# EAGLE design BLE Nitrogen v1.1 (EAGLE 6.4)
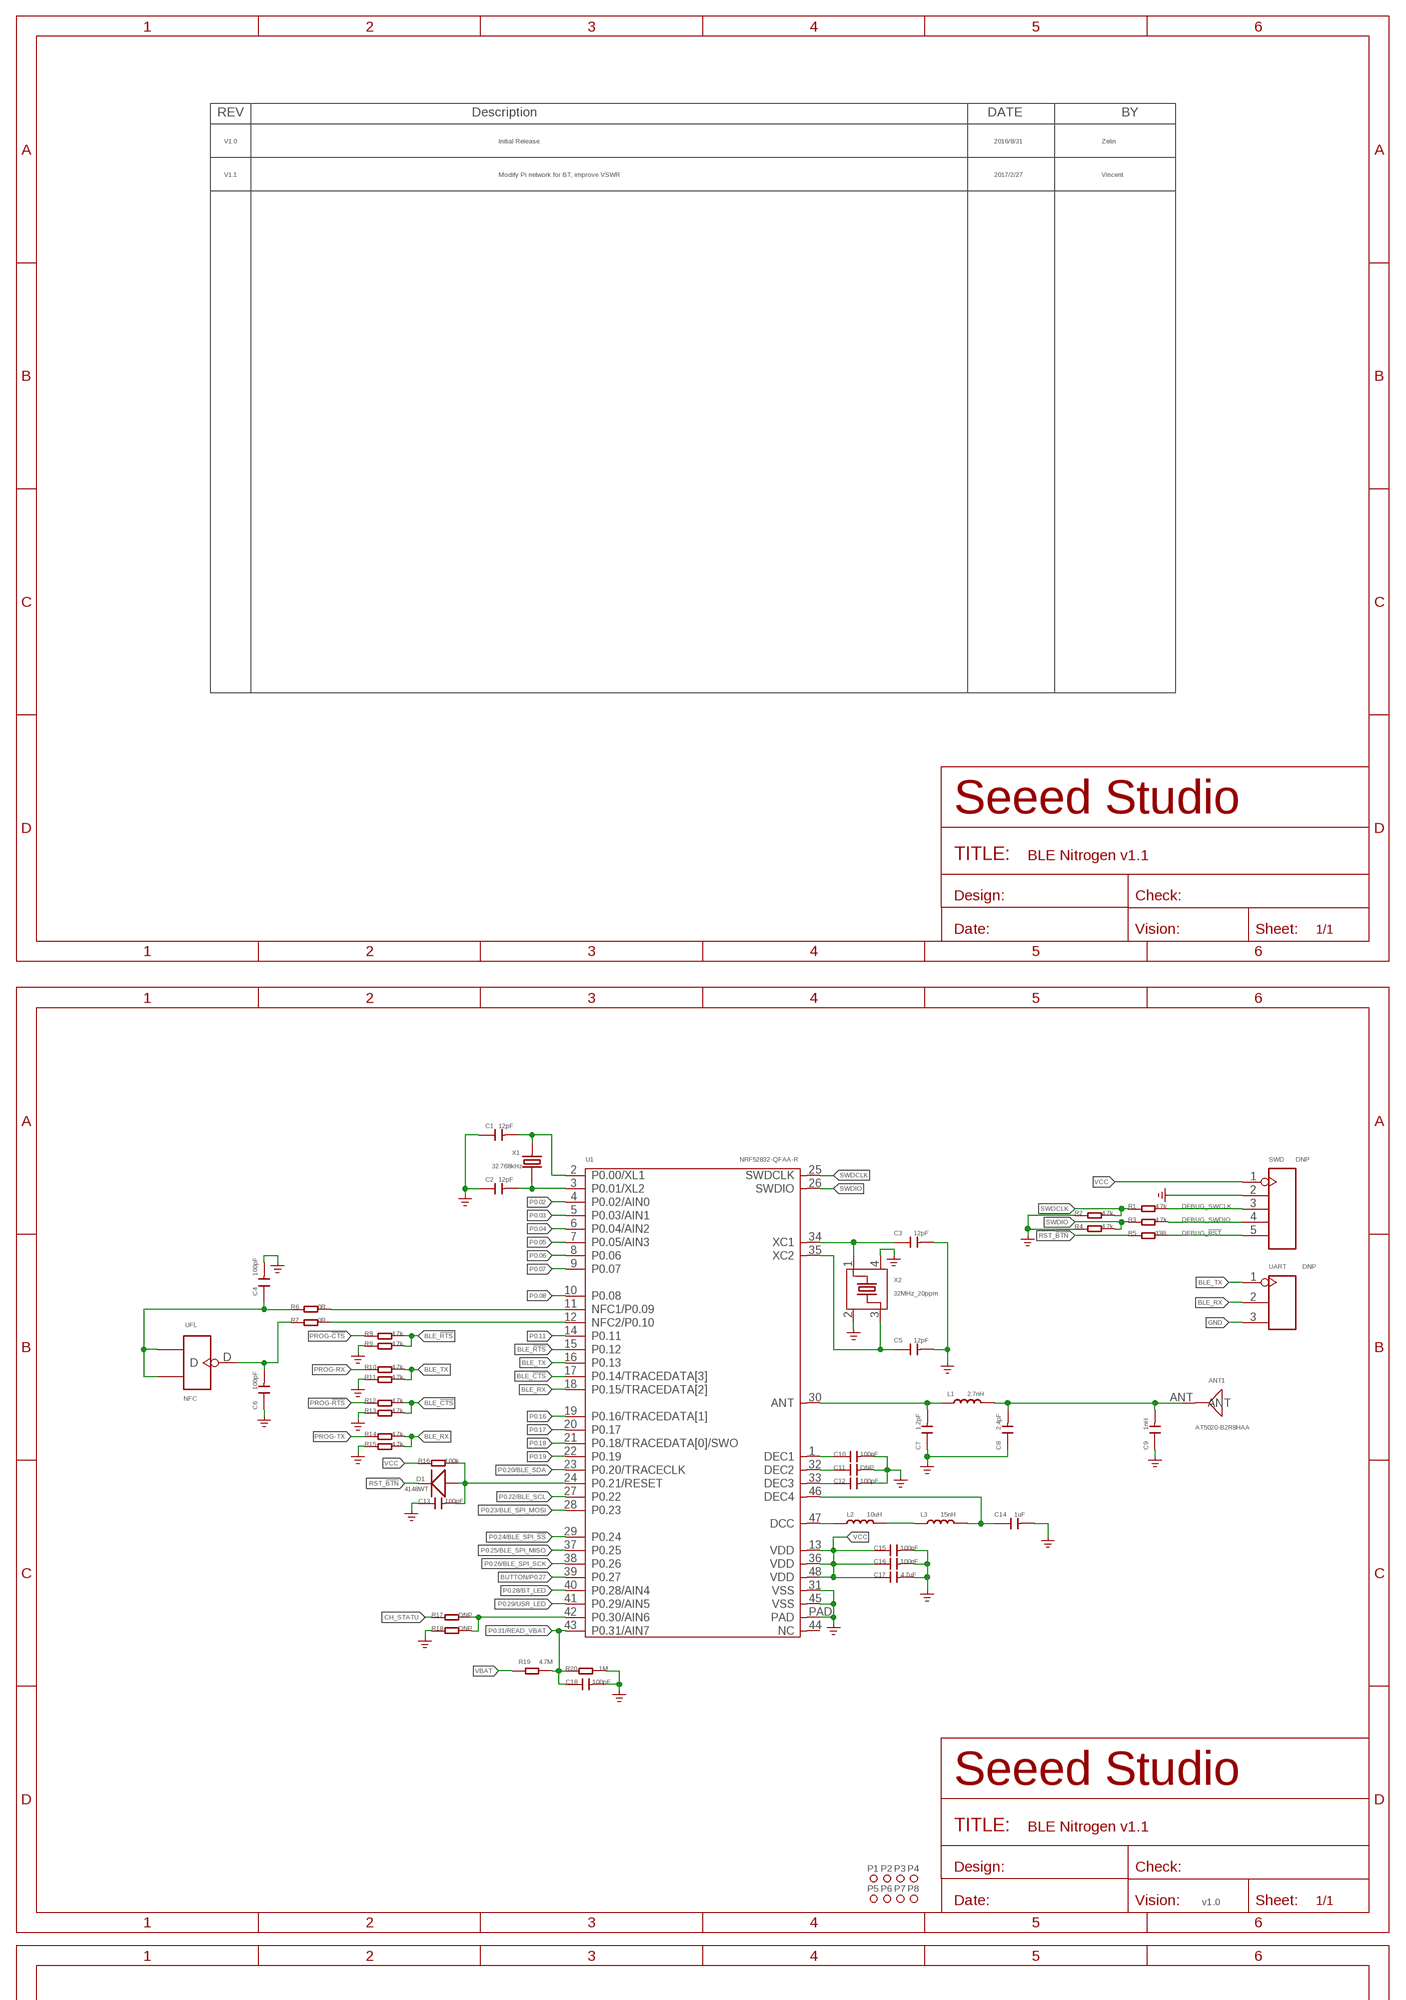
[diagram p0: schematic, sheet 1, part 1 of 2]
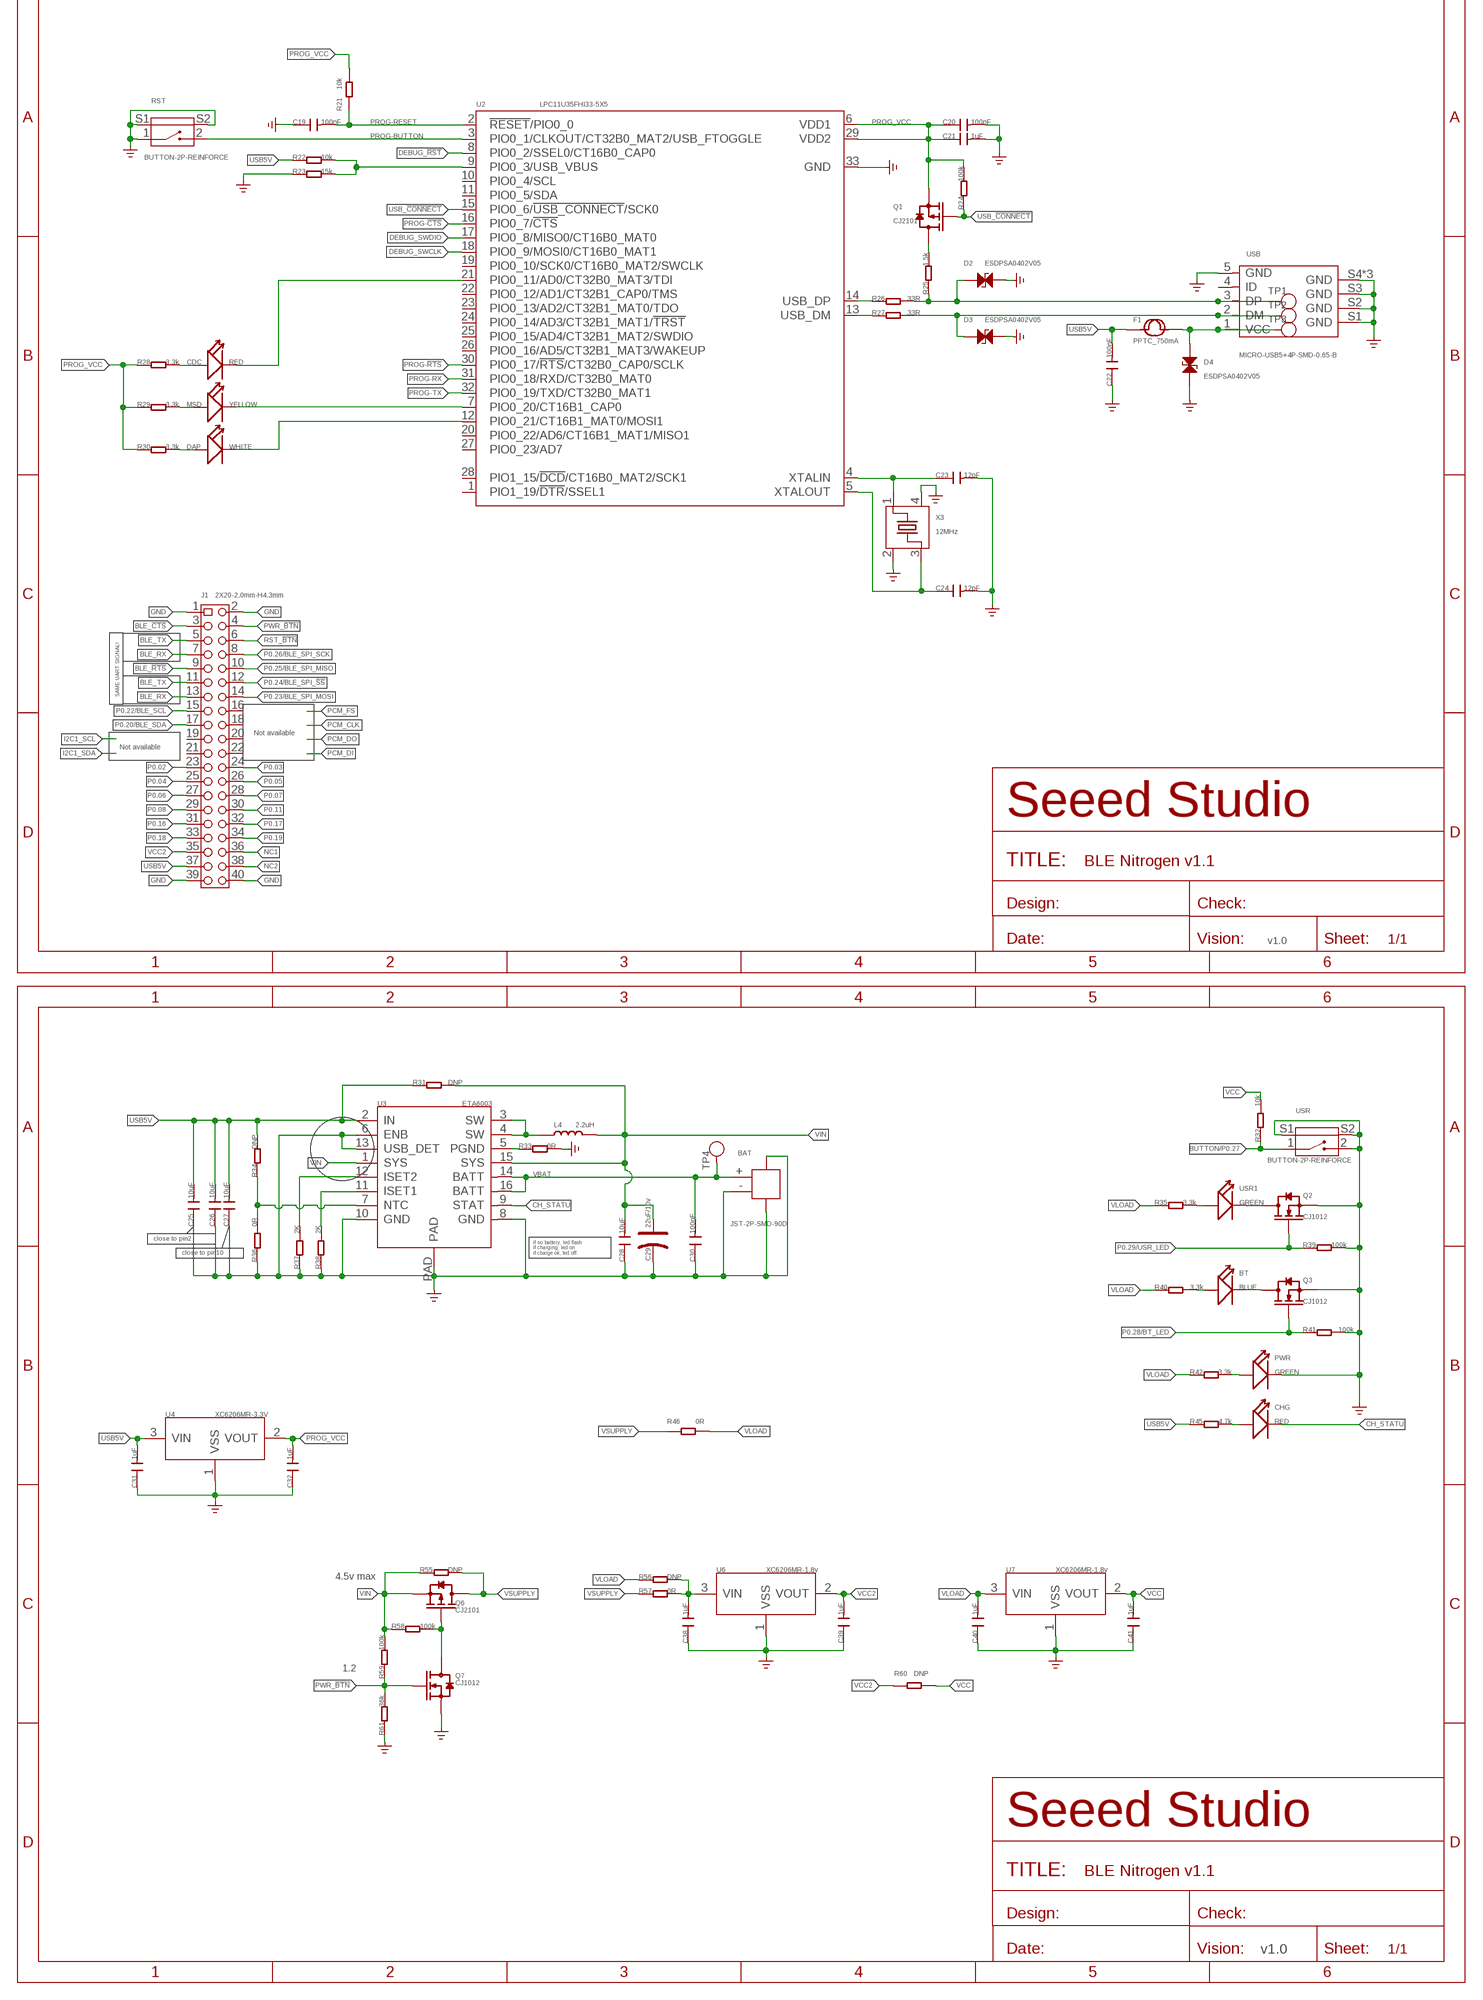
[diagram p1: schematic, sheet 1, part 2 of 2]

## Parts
ANT1  AT5020-B2R8HAA  ANTENNA-AN2051-2.4G  [ANT-SMD2P-5.05X2X1.07MM]
BAT  JST-2P-SMD-90D  JST-2P-SMD'1.0'  [HW2-SMD-1.0-90D]
BT  BLUE  LED'0402'  [LED-0402]
C1  12pF  C-0402  [C0402]
C2  12pF  C-0402  [C0402]
C3  12pF  C-0402  [C0402]
C4  100pF  C-0402  [C0402]
C5  12pF  C-0402  [C0402]
C6  100pF  C-0402  [C0402]
C7  1.2pF  C-0402  [C0402]
C8  2.4pF  C-0402  [C0402]
C9  1nH  C-0402  [C0402]
C10  100nF  C-0402  [C0402]
C11  DNP  C-0402  [C0402]
C12  100pF  C-0402  [C0402]
C13  100pF  C-0402  [C0402]
C14  1uF  C-0402  [C0402]
C15  100nF  C-0402  [C0402]
C16  100nF  C-0402  [C0402]
C17  4.7uF  C-0402  [C0402]
C18  100pF  C-0402  [C0402]
C19  100nF  C-0402  [C0402]
C20  100nF  C-0402  [C0402]
C21  1uF  C-0402  [C0402]
C22  100nF  C-0402  [C0402]
C23  12pF  C-0402  [C0402]
C24  12pF  C-0402  [C0402]
C25  10uF  C-0603  [C0603]
C26  10uF  C-0603  [C0603]
C27  10uF  C-0603  [C0603]
C28  10uF  C-0603  [C0603]
C29  22uF/10v  CAP-POLAR-AVX-A  [AVX-A]
C30  100nF  C-0402  [C0402]
C31  1uF  C-0603  [C0603]
C32  1uF  C-0603  [C0603]
C38  1uF  C-0603  [C0603]
C39  1uF  C-0603  [C0603]
C40  1uF  C-0603  [C0603]
C41  1uF  C-0603  [C0603]
CDC  RED  LED'0402'  [LED-0402]
CHG  RED  LED'0402'  [LED-0402]
D1  4148WT  D'0603'  [SOD523]
D2  ESDPSA0402V05  D-ESD-2P-DOUBLE  [ESD-0402]
D3  ESDPSA0402V05  D-ESD-2P-DOUBLE  [ESD-0402]
D4  ESDPSA0402V05  D-ESD-2P-DOUBLE  [ESD-0402]
DAP  WHITE  LED'0402'  [LED-0402]
F1  PPTC_750mA  FUSE'1206'  [F1206]
J1  2X20-2.0mm-H4.3mm  HEADER-2X20P-2.0  [H2X20-2.0]
L1  2.7nH  L'0402'  [L0402]
L2  10uH  L'0603'  [L0603]
L3  15nH  L'0402'  [L0402]
L4  2.2uH  L'0805'  [L0805]
MSD  YELLOW  LED'0402'  [LED-0402]
NFC  UFL  ANTENNA-U-FL  [U-FL3P-SMD-2.6X2.6X1.0MM]
P1  MARK-1.0'ANNULAR'  [ROUND-MARK-1.0]
P2  MARK-1.0'ANNULAR'  [ROUND-MARK-1.0]
P3  MARK-1.0'ANNULAR'  [ROUND-MARK-1.0]
P4  MARK-1.0'ANNULAR'  [ROUND-MARK-1.0]
P5  MARK-1.0'ANNULAR'  [ROUND-MARK-1.0]
P6  MARK-1.0'ANNULAR'  [ROUND-MARK-1.0]
P7  MARK-1.0'ANNULAR'  [ROUND-MARK-1.0]
P8  MARK-1.0'ANNULAR'  [ROUND-MARK-1.0]
PWR  GREEN  LED'0402'  [LED-0402]
Q1  CJ2101  MOSFET-P-SOT323  [SOT323]
Q2  CJ1012  MOSFET-N-SOT523  [SOT523]
Q3  CJ1012  MOSFET-N-SOT523  [SOT523]
Q6  CJ2101  MOSFET-P-SOT323  [SOT323]
Q7  CJ1012  MOSFET-N-SOT523  [SOT523]
R1  4.7k  R-0402  [R0402]
R2  4.7k  R-0402  [R0402]
R3  4.7k  R-0402  [R0402]
R4  4.7k  R-0402  [R0402]
R5  33R  R-0402  [R0402]
R6  0R  R-0402  [R0402]
R7  0R  R-0402  [R0402]
R8  4.7k  R-0402  [R0402]
R9  4.7k  R-0402  [R0402]
R10  4.7k  R-0402  [R0402]
R11  4.7k  R-0402  [R0402]
R12  4.7k  R-0402  [R0402]
R13  4.7k  R-0402  [R0402]
R14  4.7k  R-0402  [R0402]
R15  4.7k  R-0402  [R0402]
R16  100k  R-0402  [R0402]
R17  DNP  R-0402  [R0402]
R18  DNP  R-0402  [R0402]
R19  4.7M  R-0402  [R0402]
R20  1M  R-0402  [R0402]
R21  10k  R-0402  [R0402]
R22  10k  R-0402  [R0402]
R23  15k  R-0402  [R0402]
R24  100k  R-0402  [R0402]
R25  1.5k  R-0402  [R0402]
R26  33R  R-0402  [R0402]
R27  33R  R-0402  [R0402]
R28  3.3k  R-0402  [R0402]
R29  3.3k  R-0402  [R0402]
R30  3.3k  R-0402  [R0402]
R31  DNP  R-0402  [R0402]
R32  10k  R-0402  [R0402]
R33  0R  R-0402  [R0402]
R34  DNP  R-0402  [R0402]
R35  3.3k  R-0402  [R0402]
R36  0R  R-0402  [R0402]
R37  2K  R-0402  [R0402]
R38  2K  R-0402  [R0402]
R39  100k  R-0402  [R0402]
R40  3.3k  R-0402  [R0402]
R41  100k  R-0402  [R0402]
R42  3.3k  R-0402  [R0402]
R45  4.7k  R-0402  [R0402]
R46  0R  R-0603  [R0603]
R55  DNP  R-0402  [R0402]
R56  DNP  R-0402  [R0402]
R57  0R  R-0402  [R0402]
R58  100k  R-0402  [R0402]
R59  100k  R-0402  [R0402]
R60  DNP  R-0402  [R0402]
R61  36k  R-0402  [R0402]
RST  BUTTON-2P-REINFORCE  [4P-SMD-4.7X3.5X1.8]
SWD  DNP  HEADER-5P-2.54  [H5-2.54]
TP1  DP  TEST-POINT'4545'  [TP-D45MIL]
TP2  DM  TEST-POINT'4545'  [TP-D45MIL]
TP3  VBUS  TEST-POINT'4545'  [TP-D45MIL]
TP4  VBAT  TEST-POINT'4545'  [TP-D45MIL]
U1  NRF52832-QFAA-R  NRF52832  [QFN48-6X6MM]
U2  LPC11U35FHI33-5X5  [HVQFN33]
U3  ETA6003  PMIC-ETA6003  [QFN16G-0.5-3X3MM]
U4  XC6206MR-3.3V  XC6206MR  [SOT23]
U6  XC6206MR-1.8v  XC6206MR  [SOT23]
U7  XC6206MR-1.8v  XC6206MR  [SOT23]
UART  DNP  HEADER-3P-2.54  [H3-2.54]
USB  MICRO-USB5+4P-SMD-0.65-B  MICRO-USB5+4P'5+4P'  [MICRO-USB5+4P-SMD-0.65-B]
USR  BUTTON-2P-REINFORCE  [4P-SMD-4.7X3.5X1.8]
USR1  GREEN  LED'0402'  [LED-0402]
X1  32.768kHz  CRYSTAL-3215  [2P-SMD-3.2X1.5]
X2  32MHz_20ppm  CRYSTAL-4P  [X4-SMD-3.2X2.5X0.7MM]
X3  12MHz  CRYSTAL-4P  [X4-SMD-3.2X2.5X0.7MM]

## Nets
!RESET: C13.2 D1.+ R16.2 U1.24(P0.21/RESET)
BLE_!CTS: J1.3 R12.2 R13.2 U1.17(P0.14/TRACEDATA[3])
BLE_!RTS: J1.9 R8.2 R9.2 U1.15(P0.12)
BLE_RX: J1.7 J1.13 R14.2 R15.2 U1.18(P0.15/TRACEDATA[2]) UART.2
BLE_TX: J1.5 J1.11 R10.2 R11.2 U1.16(P0.13) UART.1
BUTTON/P0.27: R32.1 U1.39(P0.27) USR.1
CH_STATU: CHG.- R17.1 U3.9(STAT)
DEBUG_!RST: R5.2 SWD.5 U2.8(PIO0_2/SSEL0/CT16B0_CAP0)
DEBUG_SWCLK: R1.2 SWD.3 U2.18(PIO0_9/MOSI0/CT16B0_MAT1)
DEBUG_SWDIO: R3.2 SWD.4 U2.17(PIO0_8/MISO0/CT16B0_MAT0)
GND: BAT.3 BAT.4 BAT.- C1.1 C2.1 C3.2 C4.2 C5.2 C6.1 C7.1 C8.1 C9.1 C10.2 C11.2 C12.2 C13.1 C14.2 C15.2 C16.2 C17.2 C18.2 C19.1 C20.2 C21.2 C22.1 C23.2 C24.2 C25.1 C26.1 C27.1 C28.1 C29.- C30.1 C31.1 C32.1 C38.1 C39.1 C40.1 C41.1 D2.2 D3.2 D4.1 J1.1 J1.2 J1.39 J1.40 PWR.- Q2.2(S) Q3.2(S) Q7.2(S) R2.1 R4.1 R9.1 R11.1 R13.1 R15.1 R18.1 R20.2 R23.1 R33.2 R36.1 R37.1 R38.1 R39.2 R41.2 R61.1 RST.1 RST.S1 RST.S2 SWD.2 U1.31(VSS) U1.45(VSS) U1.PAD U2.33(GND) U3.6(ENB) U3.8(GND) U3.10(GND) U3.13(USB_DET) U3.PAD U4.1(VSS) U6.1(VSS) U7.1(VSS) UART.3 USB.5(GND) USB.S1(GND) USB.S2(GND) USB.S3(GND) USB.S4(GND) USB.S5(GND) USB.S6(GND) USR.2 USR.S1 USR.S2 X2.2 X2.4 X3.2 X3.4 ; supply symbol labelled GND_POWER
N$1: C4.1 NFC.GND1 NFC.GND2 R6.1
N$2: C23.1 U2.4(XTALIN) X3.1
N$3: C14.1 L3.2 U1.46(DEC4)
N$4: C24.1 U2.5(XTALOUT) X3.3
N$5: L2.1 U1.47(DCC)
N$6: R26.1 U2.14(USB_DP)
N$7: R27.1 U2.13(USB_DM)
N$8: D2.1 R25.1 R26.2 TP1.T USB.3(DP)
N$9: CHG.+ R45.2
N$10: Q6.1(G) Q7.3(D) R58.2
N$11: D3.1 R27.2 TP2.T USB.2(DM)
N$12: C1.2 U1.2(P0.00/XL1) X1.2
N$13: C2.2 U1.3(P0.01/XL2) X1.1
N$14: C3.1 U1.34(XC1) X2.1
N$15: C5.1 U1.35(XC2) X2.3
N$16: CDC.- U2.21(PIO0_11/AD0/CT32B0_MAT3/TDI)
N$17: C6.2 NFC.D R7.1
N$18: R6.2 U1.11(NFC1/P0.09)
N$19: C10.1 U1.1(DEC1)
N$20: C11.1 U1.32(DEC2)
N$21: C12.1 U1.33(DEC3)
N$22: R7.2 U1.12(NFC2/P0.10)
N$25: C7.2 L1.1 U1.30(ANT)
N$26: ANT1.ANT C8.2 C9.2 L1.2
N$28: C38.2 R56.2 R57.2 U6.3(VIN)
N$32: L2.2 L3.1
N$33: R35.2 USR1.+
N$34: BT.+ R40.2
N$35: Q2.3(D) USR1.-
N$36: BT.- Q3.3(D)
N$39: Q1.3(D) R25.2
N$40: D4.2 F1.2 TP3.T USB.1(VCC)
N$41: R22.2 R23.2 U2.9(PIO0_3/USB_VBUS)
N$42: CDC.+ R28.2
N$43: DAP.+ R30.2
N$44: MSD.+ R29.2
N$46: MSD.- U2.7(PIO0_20/CT16B1_CAP0)
N$47: DAP.- U2.12(PIO0_21/CT16B1_MAT0/MOSI1)
N$58: PWR.+ R42.2
N$84: L4.1 U3.3(SW) U3.4(SW)
N$88: R34.1 R36.2 U3.7(NTC)
N$89: R38.2 U3.11(ISET1)
N$90: R37.2 U3.12(ISET2)
N$91: R33.1 U3.5(PGND)
NC1: J1.36
NC2: J1.38
P0.02: J1.23 U1.4(P0.02/AIN0)
P0.03: J1.24 U1.5(P0.03/AIN1)
P0.04: J1.25 U1.6(P0.04/AIN2)
P0.05: J1.26 U1.7(P0.05/AIN3)
P0.06: J1.27 U1.8(P0.06)
P0.07: J1.28 U1.9(P0.07)
P0.08: J1.29 U1.10(P0.08)
P0.11: J1.30 U1.14(P0.11)
P0.16: J1.31 U1.19(P0.16/TRACEDATA[1])
P0.17: J1.32 U1.20(P0.17)
P0.18: J1.33 U1.21(P0.18/TRACEDATA[0]/SWO)
P0.19: J1.34 U1.22(P0.19)
P0.20/BLE_SDA: J1.17 U1.23(P0.20/TRACECLK)
P0.22/BLE_SCL: J1.15 U1.27(P0.22)
P0.23/BLE_SPI_MOSI: J1.14 U1.28(P0.23)
P0.24/BLE_SPI_!SS: J1.12 U1.29(P0.24)
P0.25/BLE_SPI_MISO: J1.10 U1.37(P0.25)
P0.26/BLE_SPI_SCK: J1.8 U1.38(P0.26)
P0.28/BT_LED: Q3.1(G) R41.1 U1.40(P0.28/AIN4)
P0.29/USR_LED: Q2.1(G) R39.1 U1.41(P0.29/AIN5)
P0.30/AIN6: R17.2 R18.2 U1.42(P0.30/AIN6)
P0.31/READ_VBAT: C18.1 R19.2 R20.1 U1.43(P0.31/AIN7)
PROG-!CTS!: R8.1 U2.16(PIO0_7/!CTS!)
PROG-!RTS!: R12.1 U2.30(PIO0_17/!RTS!/CT32B0_CAP0/SCLK)
PROG-BUTTON: RST.2 U2.3(PIO0_1/CLKOUT/CT32B0_MAT2/USB_FTOGGLE)
PROG-RESET: C19.2 R21.1 U2.2(!RESET!/PIO0_0)
PROG-RX: R10.1 U2.31(PIO0_18/RXD/CT32B0_MAT0)
PROG-TX: R14.1 U2.32(PIO0_19/TXD/CT32B0_MAT1)
PROG_VCC: C20.1 C21.1 C32.2 Q1.2(S) R21.2 R24.2 R28.1 R29.1 R30.1 U2.6(VDD1) U2.29(VDD2) U4.2(VOUT)
PWR_!BTN: J1.4 Q7.1(G) R59.1 R61.2
RST_!BTN: D1.- J1.6 R5.1
SWDCLK: R1.1 R2.2 U1.25(SWDCLK)
SWDIO: R3.1 R4.2 U1.26(SWDIO)
USB5V: C22.2 C25.2 C26.2 C27.2 C31.2 F1.1 J1.37 R22.1 R31.1 R34.2 R45.1 U3.2(IN) U4.3(VIN)
USB_!CONNECT!: Q1.1(G) R24.1 U2.15(PIO0_6/!USB_CONNECT!/SCK0)
VBAT: BAT.+ C30.2 R19.1 TP4.T U3.14(BATT) U3.16(BATT)
VCC: C15.1 C16.1 C17.1 C41.2 R16.1 R32.2 R60.1 SWD.1 U1.13(VDD) U1.36(VDD) U1.48(VDD) U7.2(VOUT)
VCC2: C39.2 J1.35 R60.2 U6.2(VOUT)
VIN: C28.2 C29.+ L4.2 Q6.2(S) R31.2 R55.1 R58.1 R59.2 U3.1(SYS) U3.15(SYS)
VLOAD: C40.2 R35.1 R40.1 R42.1 R46.2 R56.1 U7.3(VIN)
VSUPPLY: Q6.3(D) R46.1 R55.2 R57.1
Unconnected: J1.16 J1.18 J1.19 J1.20 J1.21 J1.22 U1.44(NC) U2.1(PIO1_19/!DTR!/SSEL1) U2.10(PIO0_4/SCL) U2.11(PIO0_5/SDA) U2.19(PIO0_10/SCK0/CT16B0_MAT2/SWCLK) U2.20(PIO0_22/AD6/CT16B1_MAT1/MISO1) U2.22(PIO0_12/AD1/CT32B1_CAP0/TMS) U2.23(PIO0_13/AD2/CT32B1_MAT0/TDO) U2.24(PIO0_14/AD3/CT32B1_MAT1/!TRST!) U2.25(PIO0_15/AD4/CT32B1_MAT2/SWDIO) U2.26(PIO0_16/AD5/CT32B1_MAT3/WAKEUP) U2.27(PIO0_23/AD7) U2.28(PIO1_15/!DCD!/CT16B0_MAT2/SCK1) USB.4(ID)

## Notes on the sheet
- V1.0 | Initial Release. | 2016/8/31 | Zelin
- V1.1 | Modify Pi network for BT, improve VSWR | 2017/2/27 | Vincent
- v1.0
- SAME UART SIGNAL!
- Not available
- Not available
- v1.0
- close to pin2
- close to pin10
- if no battery, led flash.
  if charging, led on.
  if charge ok, led off.
- 4.5v max
- 1.2
- v1.0

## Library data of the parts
ANT1 = Connector-new:ANTENNA-AN2051-2.4G: Multilayer Chip Antenna for 2.4GHz Wireless Communication
BAT = Connector-update:JST-2P-SMD: 2P-SMD-1.0-90D:320110054;2P-SMD-2.0-90D:320110026
BT CDC CHG DAP MSD PWR USR1 = Discrete:LED*
C1-C28 C30-C32 C38-C41 = Discrete:C*: Ceramic Capacitors
C29 = Discrete-new:CAP-POLAR: Electrolytic Capacitors,Tantalum Capacitors and Super Capacitors
D1 = Discrete:D*
D2-D4 = Discrete-new:D-ESD-2P-DOUBLE
F1 = Discrete:FUSE
J1 = Connector-update:HEADER-2X20P-2.0
L1-L4 = Discrete:L*
NFC = Connector-update:ANTENNA-U-FL: 320110048
P1-P8 = Discrete-new:MARK-1.0; PARTNO: DNP
Q1 Q6 = Discrete:MOSFET-P
Q2 Q3 Q7 = Discrete:MOSFET-N: IRLL014: http://www.vishay.com/docs/91319/sihll014.pdf
R1-R42 R45 R46 R55-R61 = Discrete:R*
RST USR = Discrete:BUTTON-2P-REINFORCE: TS-1188E http://www.best-dz.com/?thread-374-2.html SMD Button
SWD = Connector-update:HEADER-5P
TP1-TP4 = Discrete-new:TEST-POINT; PARTNO: DNP
U1 = AMLib:NRF52832
U2 = AMLib:LPC11U35FHI33
U3 = AMLib_New:PMIC-ETA6003: 2.5A,3MHZ Switching Charger with Dynamic Power Path Management
U4 U6 U7 = IC:XC6206: LOW ESR Cap.Compatible Positive Voltage Regulators
UART = Connector-update:HEADER-3P
USB = Connector-new:MICRO-USB5+4P: 5+4P-SMD-0.65-B:320010000;5+2P-SMD-0.65-AB:340032001
X1 = Discrete:CRYSTAL*: CRYSTAL
X2 X3 = Discrete-new:CRYSTAL-4P

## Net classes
0 default: width 0.127 mm, drill 0.203 mm, clearance 0.152 mm

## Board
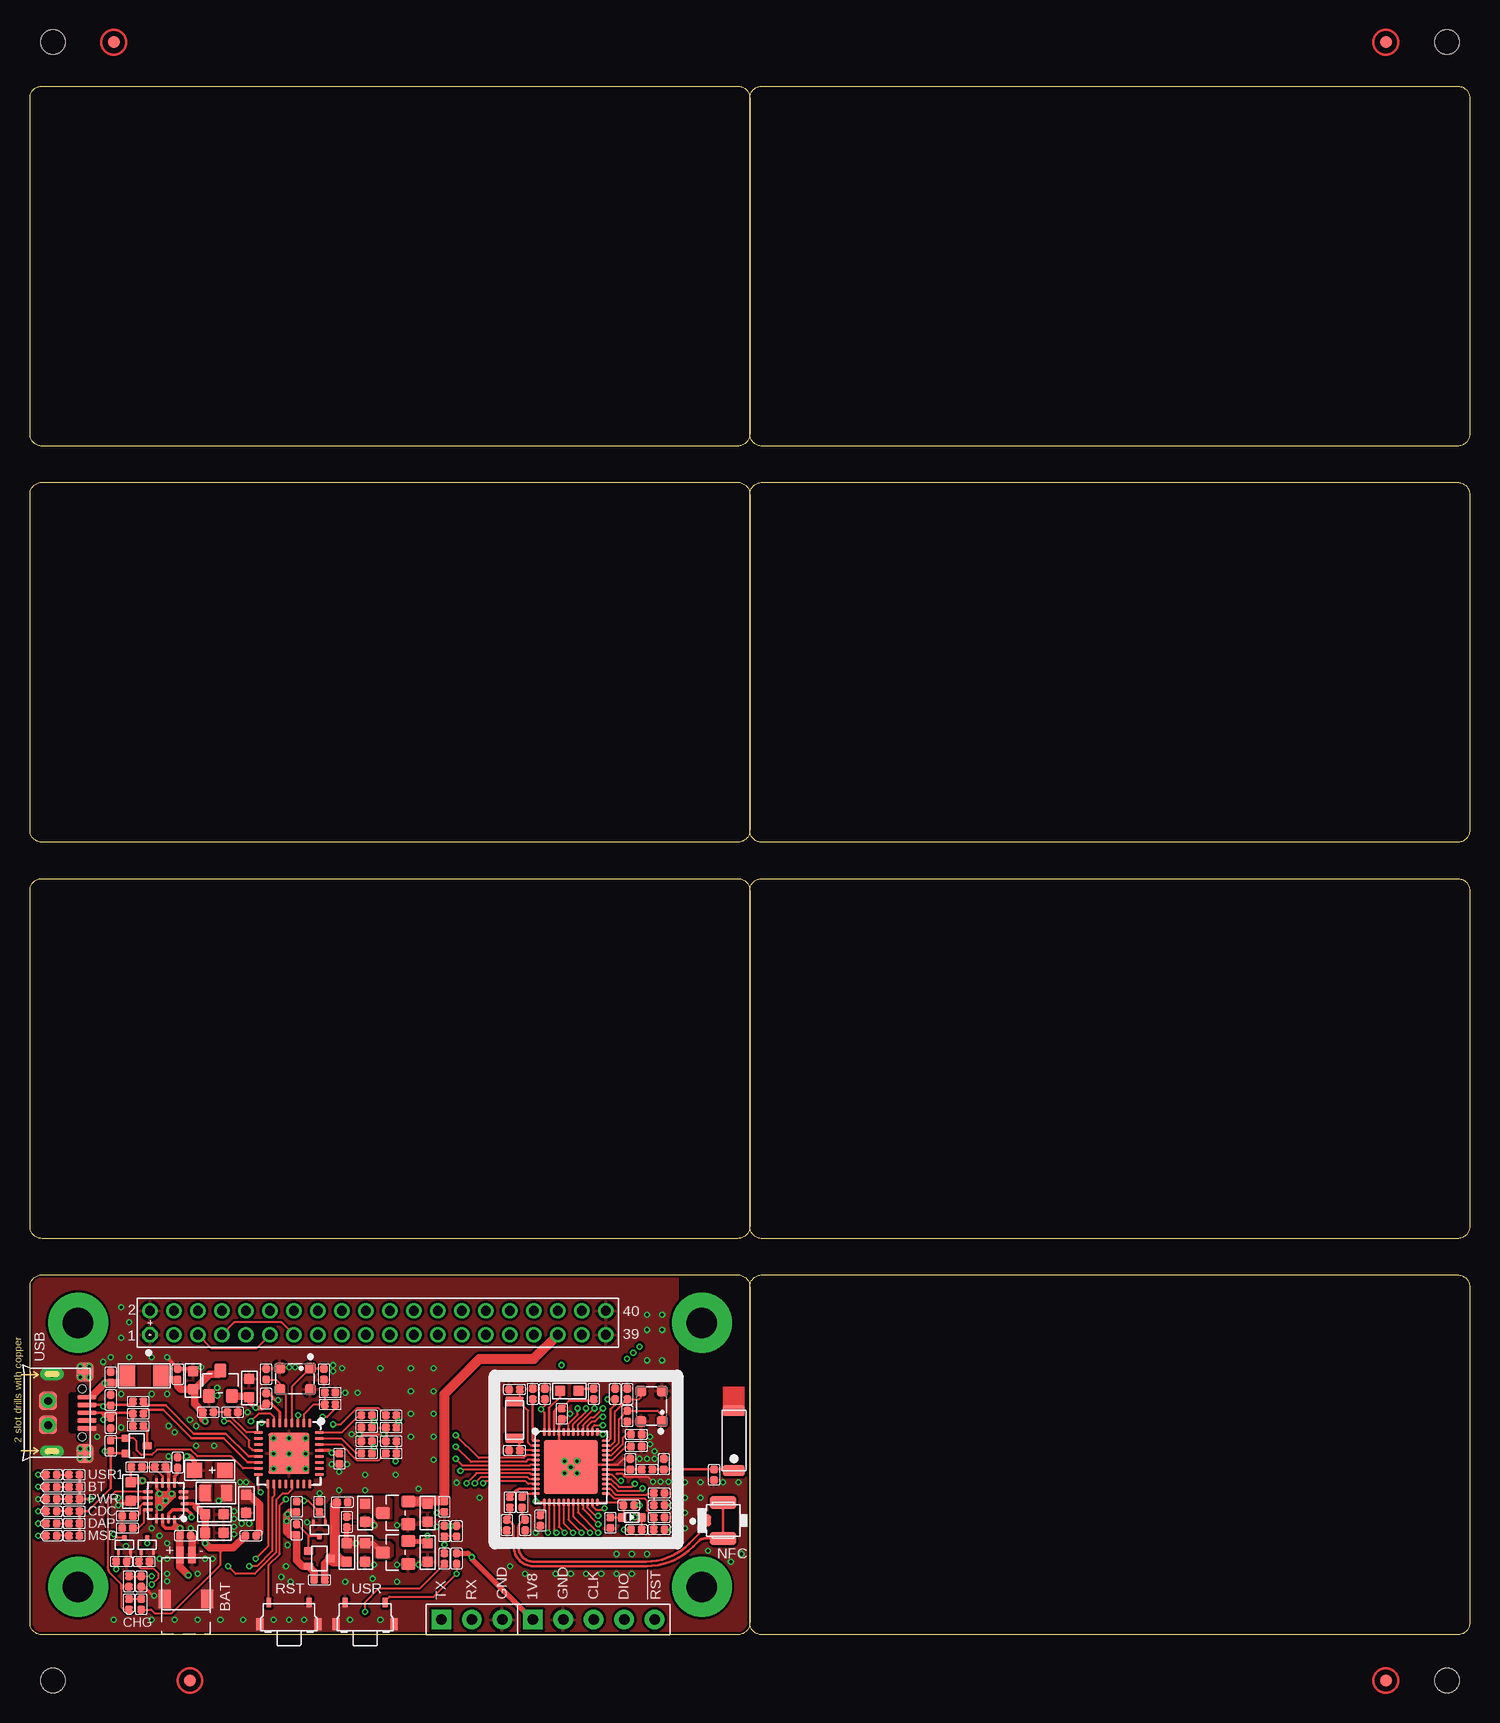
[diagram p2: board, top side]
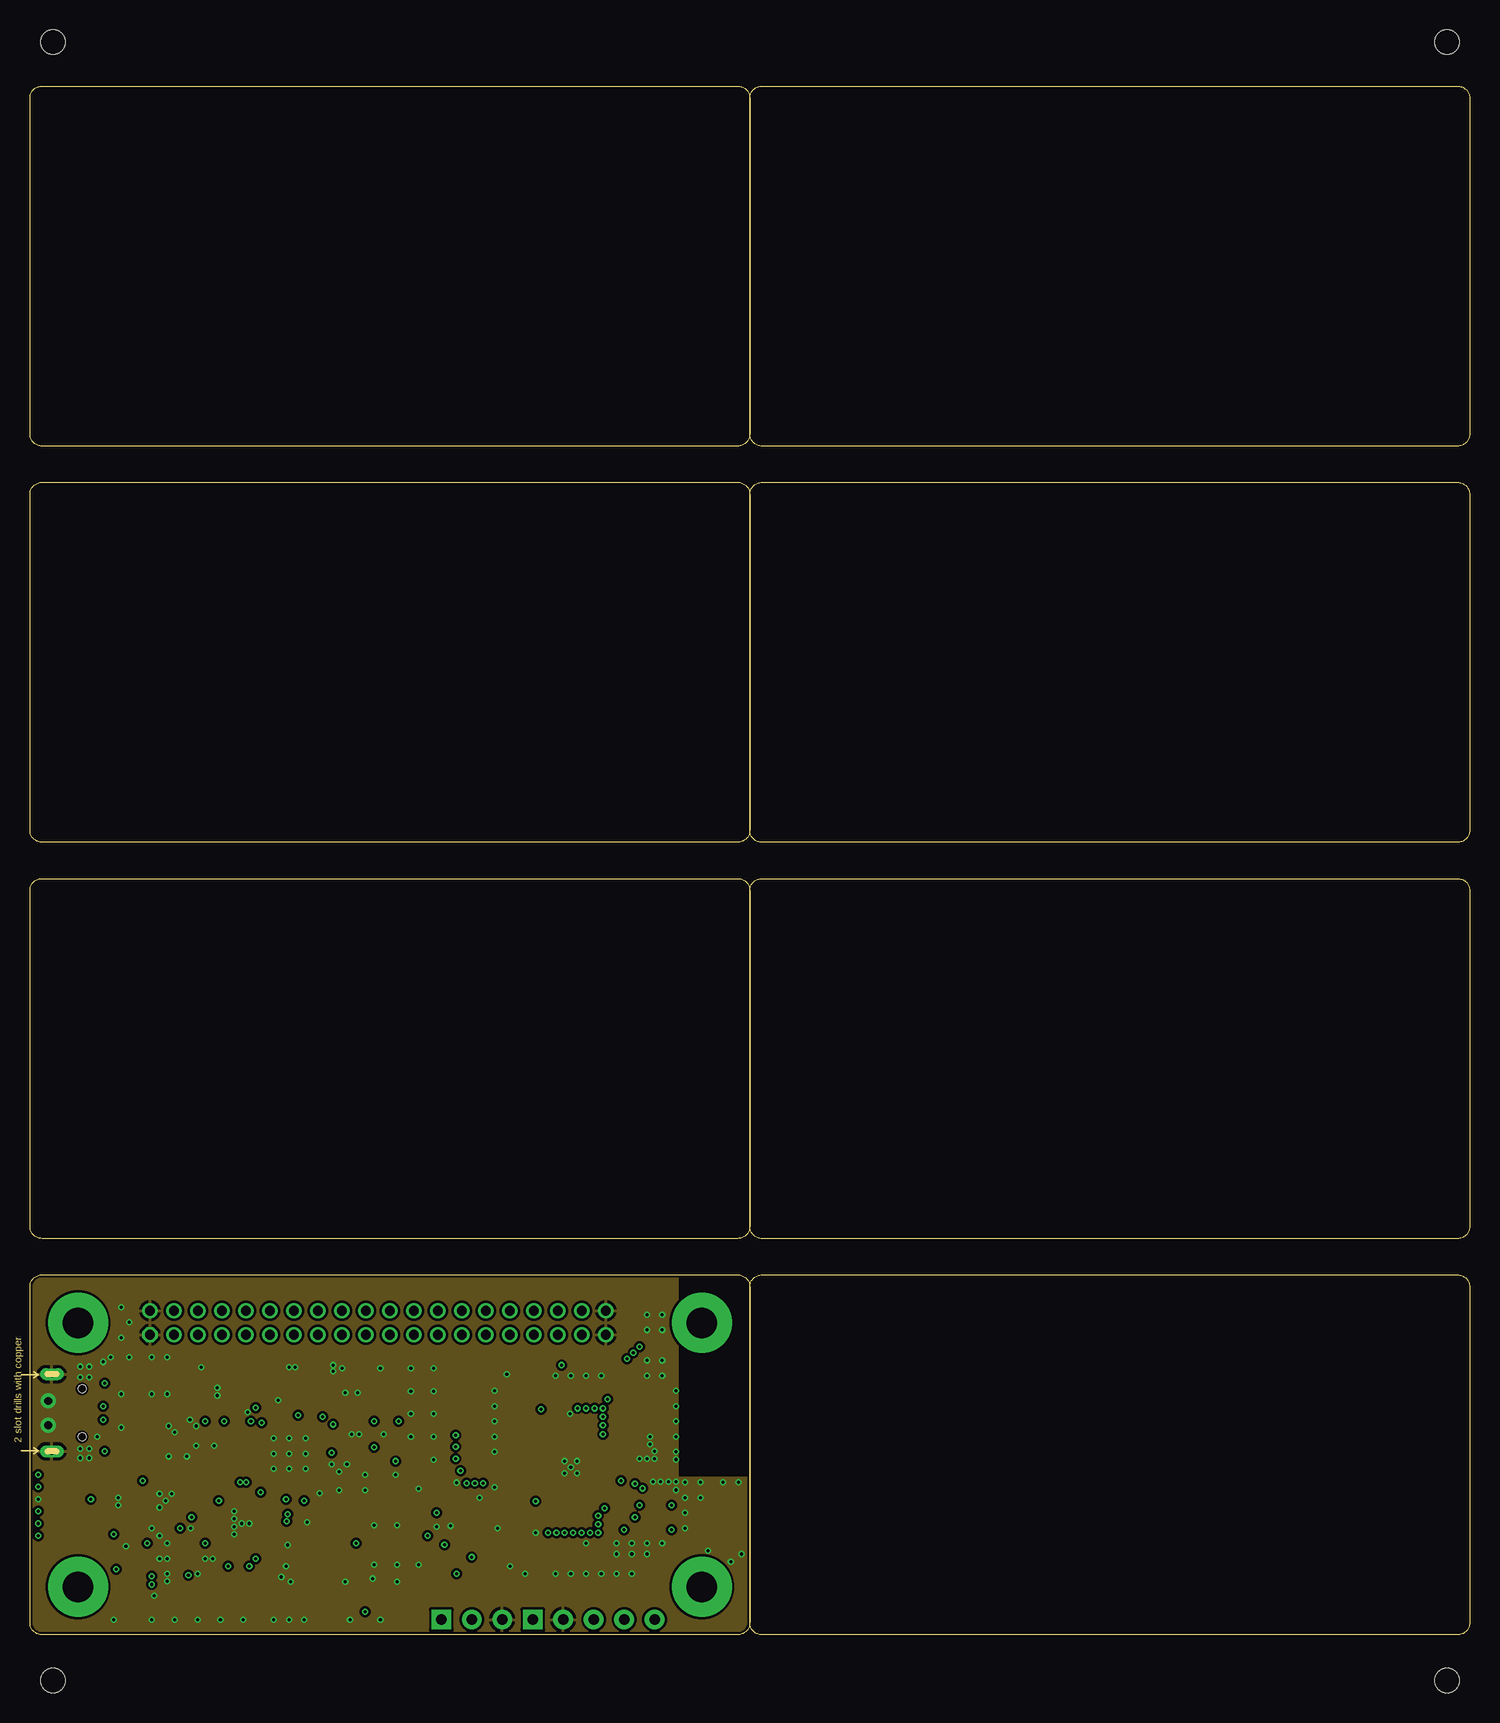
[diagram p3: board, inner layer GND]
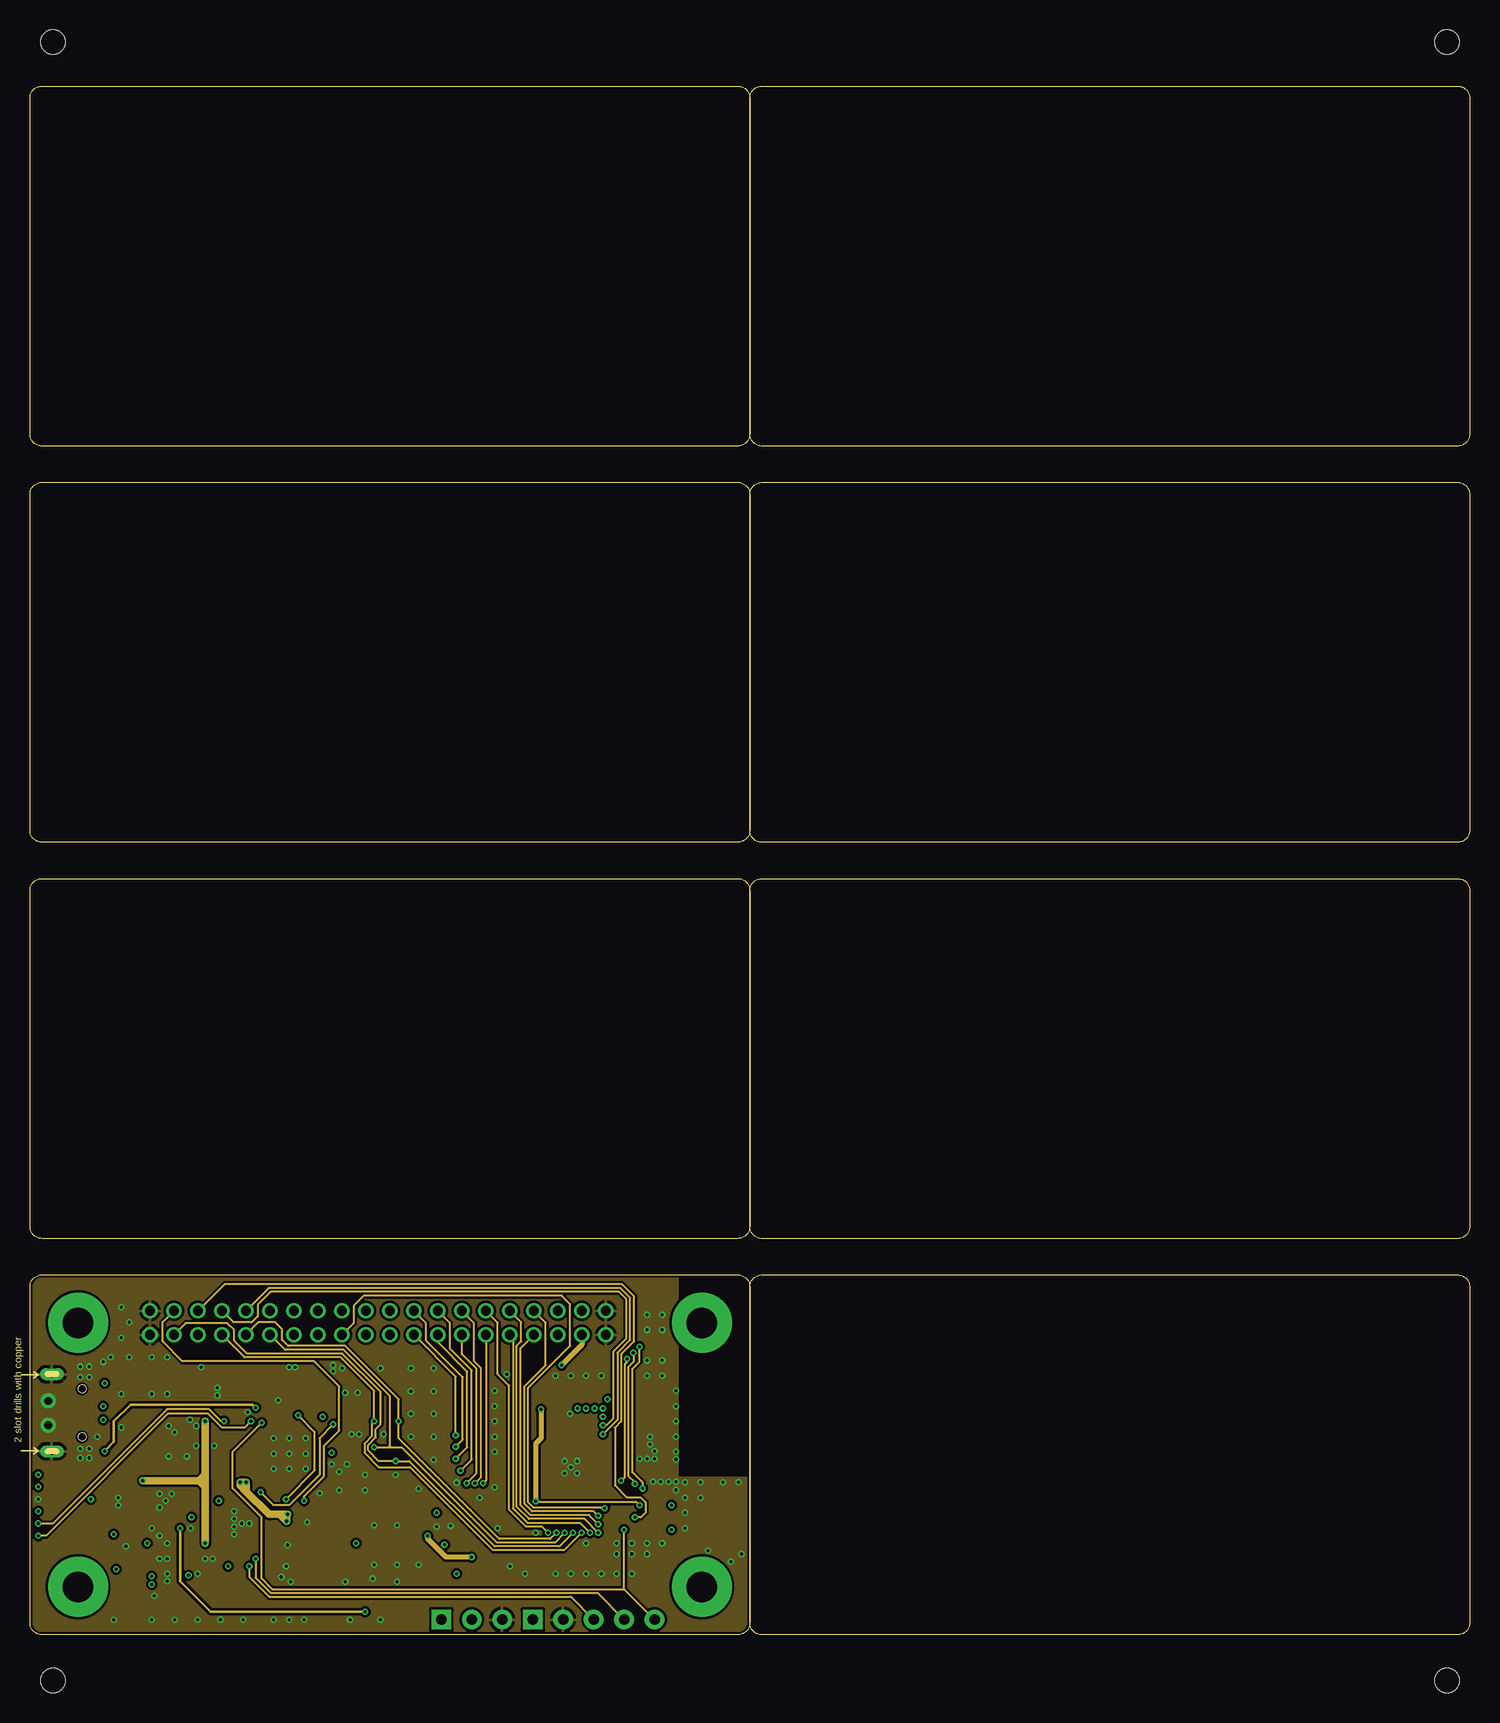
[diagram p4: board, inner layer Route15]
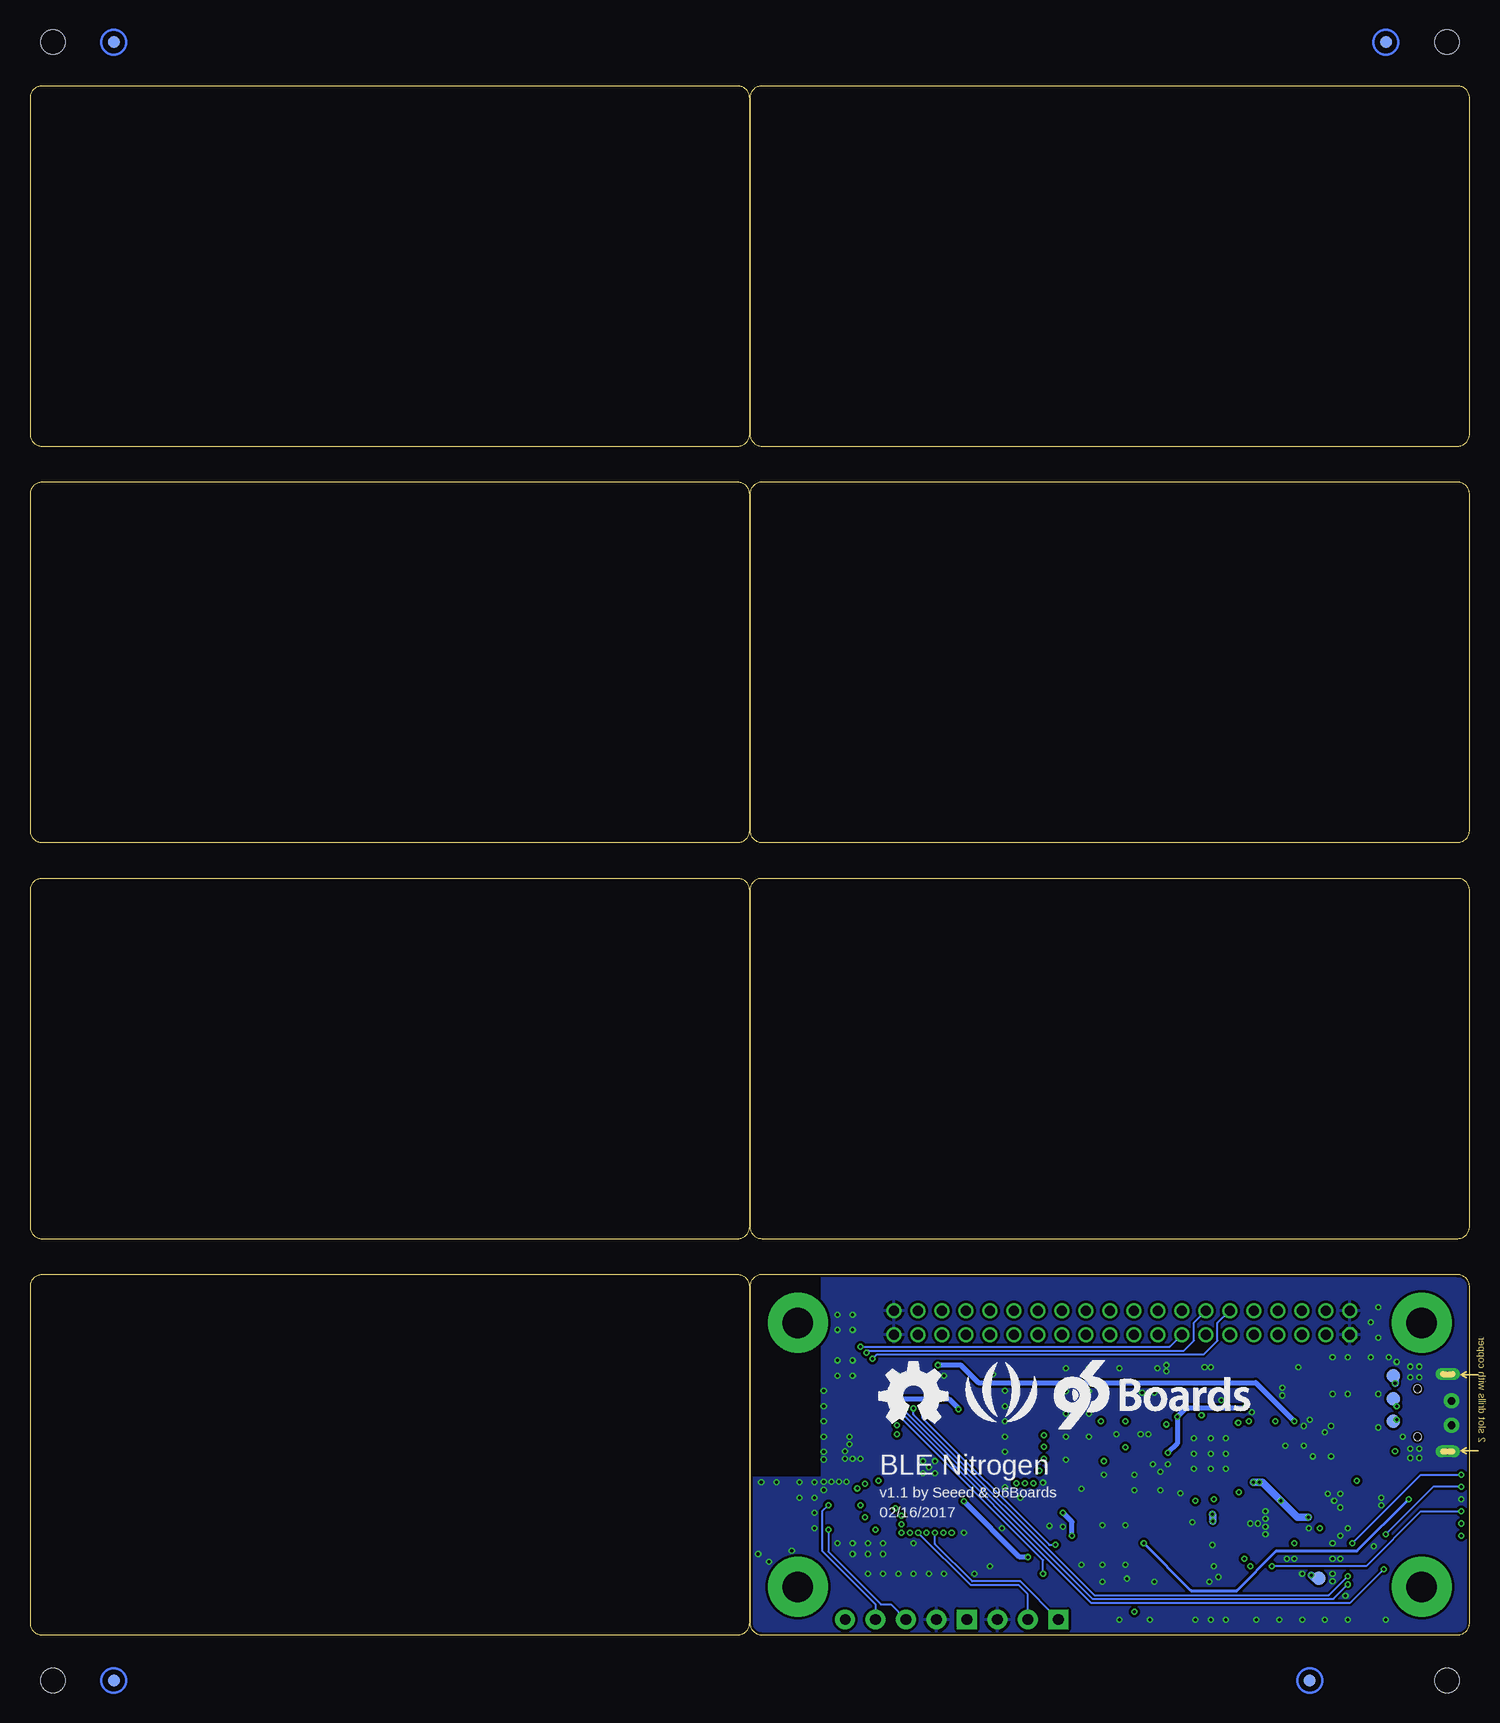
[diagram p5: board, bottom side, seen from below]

Size 120.02 x 129.06 mm. Coordinates in mm from the lower left corner, seen from the top.
Outline: 64 segments
Copper layers (1*2*15*16): Top 0.035mm / dielectric 0.2mm / GND 0.0175mm / dielectric 0.7mm / Route15 0.0175mm / dielectric 0.2mm / Bottom 0.035mm
Design rules "default *": minimum track width 6mil, minimum drill 8mil, track to track 6mil, track to pad 6mil, pad to pad 6mil, via to via 6mil, smd to smd 0mil, copper to edge 8mil, drill to drill 8mil, minimum pad ring 4mil, minimum via ring 4mil, stop-mask expansion 2mil, vias tented up to drill 20mil, thermal gap 10mil
Holes 2.03 mm at 1.91,132.72 118.11,132.72 1.91,-3.81 118.11,-3.81
tRestrict: area 42.5,11.4 to 47.6,16.5; area 10.3,10.2 to 12.3,12.2

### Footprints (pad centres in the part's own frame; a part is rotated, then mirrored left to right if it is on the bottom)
ANT-SMD2P-5.05X2X1.07MM = smd 1.8 x 0.9: ANT 0,2.513; P$1 0,-2.513
HW2-SMD-1.0-90D = smd 1.524 x 1.016: 3 -3.429,1.778; 4 -3.429,-1.778 | smd 1.397 x 0.635: + 0.254,0.508; - 0.254,-0.508
LED-0402 = smd 0.635 x 0.635: + -0.445,0; - 0.445,0
C0402 = smd 0.635 x 0.635: 1 -0.445,0; 2 0.445,0
C0603 = smd 0.889 x 0.889: 1 -0.762,0; 2 0.762,0
AVX-A = smd 1.27 x 1.27: + -1.27,0; - 1.27,0
SOD523 = smd 0.762 x 0.7: + -0.8,0; - 0.8,0
ESD-0402 = smd 0.635 x 0.635: 1 -0.445,0; 2 0.445,0
F1206 = smd 1.27 x 1.778: 1 -1.397,0; 2 1.397,0
H2X20-2.0 = drill 0.813 pad 1.27 octagon: 1 -1,0 | drill 0.813 pad 1.27: 2 1,0; 3 -1,-2; 4 1,-2; 5 -1,-4; 6 1,-4; 7 -1,-6; 8 1,-6; 9 -1,-8; 10 1,-8; 11 -1,-10; 12 1,-10; 13 -1,-12; 14 1,-12; 15 -1,-14; 16 1,-14; 17 -1,-16; 18 1,-16; 19 -1,-18; 20 1,-18; 21 -1,-20; 22 1,-20; 23 -1,-22; 24 1,-22; 25 -1,-24; 26 1,-24; 27 -1,-26; 28 1,-26; 29 -1,-28; 30 1,-28; 31 -1,-30; 32 1,-30; 33 -1,-32; 34 1,-32; 35 -1,-34; 36 1,-34; 37 -1,-36; 38 1,-36; 39 -1,-38; 40 1,-38
L0402 = smd 0.635 x 0.635: 1 -0.445,0; 2 0.445,0
L0603 = smd 0.889 x 0.889: 1 -0.762,0; 2 0.762,0
L0805 = smd 1.016 x 1.397: 1 -0.889,0; 2 0.889,0
U-FL3P-SMD-2.6X2.6X1.0MM = smd 1.05 x 1: D -1.524,0 | smd 2.2 x 1.05: GND1 0,1.5; GND2 0,-1.5
ROUND-MARK-1.0 = smd 1.016 x 1.016: P$1 0,0
SOT323 = smd 0.635 x 0.762: 1 -0.635,-0.889; 2 0.635,-0.889; 3 0,0.889
SOT523 = smd 0.305 x 0.508: 1 -0.508,-0.572; 2 0.508,-0.572 | smd 0.381 x 0.508: 3 0,0.572
R0402 = smd 0.635 x 0.635: 1 -0.445,0; 2 0.445,0
R0603 = smd 0.889 x 0.889: 1 -0.762,0; 2 0.762,0
4P-SMD-4.7X3.5X1.8 = smd 0.4 x 0.8: 1 -1.675,-1.277; 2 1.675,-1.277 | smd 0.6 x 1: S1 -2.425,0.5; S2 2.425,0.5
H5-2.54 = drill 0.889 pad 1.651 square: 1 0,5.08 | drill 0.889 pad 1.651: 2 0,2.54; 3 0,0; 4 0,-2.54; 5 0,-5.08
TP-D45MIL = smd 1.143 x 1.143: T 0,0
QFN48-6X6MM = smd 0.65 x 0.23: 1 -2.925,2.2; 2 -2.925,1.8; 3 -2.925,1.4; 4 -2.925,1; 5 -2.925,0.6; 6 -2.925,0.2; 7 -2.925,-0.2; 8 -2.925,-0.6; 9 -2.925,-1; 10 -2.925,-1.4; 11 -2.925,-1.8; 12 -2.925,-2.2; 25 2.925,-2.2; 26 2.925,-1.8; 27 2.925,-1.4; 28 2.925,-1; 29 2.925,-0.6; 30 2.925,-0.2; 31 2.925,0.2; 32 2.925,0.6; 33 2.925,1; 34 2.925,1.4; 35 2.925,1.8; 36 2.925,2.2 | smd 0.23 x 0.65: 13 -2.2,-2.925; 14 -1.8,-2.925; 15 -1.4,-2.925; 16 -1,-2.925; 17 -0.6,-2.925; 18 -0.2,-2.925; 19 0.2,-2.925; 20 0.6,-2.925; 21 1,-2.925; 22 1.4,-2.925; 23 1.8,-2.925; 24 2.2,-2.925; 37 2.2,2.925; 38 1.8,2.925; 39 1.4,2.925; 40 1,2.925; 41 0.6,2.925; 42 0.2,2.925; 43 -0.2,2.925; 44 -0.6,2.925; 45 -1,2.925; 46 -1.4,2.925; 47 -1.8,2.925; 48 -2.2,2.925 | smd 4.5 x 4.5: PAD 0,0
HVQFN33 = smd 0.762 x 0.279: 1 -2.54,1.75; 2 -2.54,1.25; 3 -2.54,0.75; 4 -2.54,0.25; 5 -2.54,-0.25; 6 -2.54,-0.75; 7 -2.54,-1.25; 8 -2.54,-1.75; 17 2.54,-1.75; 18 2.54,-1.25; 19 2.54,-0.75; 20 2.54,-0.25; 21 2.54,0.25; 22 2.54,0.75; 23 2.54,1.25; 24 2.54,1.75 | smd 0.279 x 0.762: 9 -1.75,-2.54; 10 -1.25,-2.54; 11 -0.75,-2.54; 12 -0.25,-2.54; 13 0.25,-2.54; 14 0.75,-2.54; 15 1.25,-2.54; 16 1.75,-2.54; 25 1.75,2.54; 26 1.25,2.54; 27 0.75,2.54; 28 0.25,2.54; 29 -0.25,2.54; 30 -0.75,2.54; 31 -1.25,2.54; 32 -1.75,2.54 | smd 3.429 x 3.429: 33 0,0
QFN16G-0.5-3X3MM = smd 0.65 x 0.28: 1 -1.575,0.75; 2 -1.575,0.25 | smd 0.85 x 0.28: 3 -1.475,-0.25; 4 -1.475,-0.75; 9 1.475,-0.75; 10 1.475,-0.25; 11 1.475,0.25; 12 1.475,0.75 | smd 0.28 x 0.85: 5 -0.75,-1.475; 6 -0.25,-1.475; 7 0.25,-1.475; 8 0.75,-1.475; 13 0.75,1.475; 14 0.25,1.475 | smd 0.28 x 0.65: 15 -0.25,1.575; 16 -0.75,1.575 | smd 0.508 x 0.508: PAD 0,0
SOT23 = smd 1.016 x 1.2: 1 -0.95,-1.06; 2 0.95,-1.06; 3 0,1.06
96BOARDS_IOT_EDITION_STANDARD = drill 2.54 pad 5: P$1 4,26; P$2 4,4; P$3 56,4; P$4 56,26
H3-2.54 = drill 0.889 pad 1.651 square: 1 0,2.54 | drill 0.889 pad 1.651: 2 0,0; 3 0,-2.54
MICRO-USB5+4P-SMD-0.65-B = smd 0.381 x 1.524: 1 -1.3,-0.25; 2 -0.65,-0.25; 3 0,-0.25; 4 0.65,-0.25; 5 1.3,-0.25 | smd 1.6 x 1.397: S1 -3.4,-0.427; S6 3.4,-0.427 | drill 0.508 pad 1.016 long: S2 -3.226,-3.175; S5 3.226,-3.175 | smd 1.5 x 1.5: S3 -1,-3.5; S4 1,-3.5 | hole 0.635: -2,-0.65; 2,-0.65
2P-SMD-3.2X1.5 = smd 0.762 x 1.524: 1 -1.524,0; 2 1.524,0
X4-SMD-3.2X2.5X0.7MM = smd 0.889 x 0.889: 1 -1.27,-0.889; 2 1.27,-0.889; 3 1.27,0.889; 4 -1.27,0.889

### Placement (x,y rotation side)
ANT1  58.67,16.2 180 top
BAT  13,6.4 90 top
BT  1.78,12.32 180 top
C1  40.39,20.45 0 top
C2  40.39,15.37 0 top
C3  49.78,18.23 270 top
C4  39.75,9.15 270 top
C5  49.78,20.07 90 top
C6  41.27,9.15 90 top
C7  50.04,14.23 270 top
C8  52.84,14.23 270 top
C9  57.02,13.34 90 top
C10  41.91,20.07 90 top
C11  50.55,15.69 0 top
C12  50.55,16.7 0 top
C13  48.39,9.34 90 top
C14  44.32,18.42 270 top
C15  42.55,9.53 270 top
C16  48.77,20.07 90 top
C17  42.93,20.07 90 top
C18  34.54,8.64 90 top
C19  25.02,20.2 180 top
C20  25.78,14.67 270 top
C21  19.68,19.69 90 top
C22  12.32,21.72 270 top
C23  24.51,21.72 270 top
C24  19.68,21.72 90 top
C25  15.37,10.04 180 top
C26  8.38,11.94 90 top
C27  15.37,8.51 180 top
C28  18.03,10.92 90 top
C29  14.99,13.72 180 top
C30  12.95,8.26 180 top
C31  13.59,21.21 270 top
C32  18.29,20.58 270 top
C38  27.94,10.16 90 top
C39  33.15,10.16 90 top
C40  27.94,6.86 90 top
C41  33.15,6.86 90 top
CDC  1.78,10.29 180 top
CHG  8.26,2.54 270 top
D1  50.16,9.78 0 top
D2  6.73,17.66 270 top
D3  6.73,19.56 90 top
D4  6.73,21.47 270 top
DAP  1.78,9.27 180 top
F1  9.53,21.59 180 top
J1  10,26 90 top
L1  51.44,13.78 0 top
L2  44.96,20.32 0 top
L3  46.99,20.07 270 top
L4  15.49,11.81 0 top
MSD  1.78,8.26 180 top
NFC  57.78,9.53 0 top
P1  not placed on the board
P2  not placed on the board
P3  not placed on the board
P4  not placed on the board
P5  not placed on the board
P6  not placed on the board
P7  not placed on the board
P8  not placed on the board
PWR  1.78,11.31 180 top
Q1  8.89,15.75 270 top
Q2  9.78,7.5 0 top
Q3  7.87,7.5 0 top
Q6  24.13,6.35 270 top
Q7  24.13,8.77 180 top
R1  52.45,8.77 0 top
R2  52.45,9.78 180 top
R3  52.45,10.8 0 top
R4  52.45,11.81 180 top
R5  50.55,8.77 180 top
R6  40.01,11.05 90 top
R7  41.02,11.05 90 top
R8  30.1,18.29 0 top
R9  30.1,17.27 0 top
R10  28.07,15.12 0 top
R11  28.07,16.13 0 top
R12  30.1,15.12 0 top
R13  30.1,16.13 0 top
R14  28.07,18.29 0 top
R15  28.07,17.27 0 top
R16  49.91,10.8 180 top
R17  8.26,4.45 90 top
R18  9.27,4.45 90 top
R19  34.54,6.35 90 top
R20  35.56,8.64 90 top
R21  25.02,19.18 0 top
R22  14.86,18.54 0 top
R23  16.89,18.54 180 top
R24  6.73,15.75 270 top
R25  9.02,17.4 0 top
R26  9.02,18.42 180 top
R27  9.02,19.43 180 top
R28  3.68,10.29 180 top
R29  3.68,8.26 180 top
R30  3.68,9.27 180 top
R31  18.41,8.26 0 top
R32  35.56,6.35 90 top
R33  12.32,14.35 90 top
R34  8.89,13.97 180 top
R35  3.68,13.34 180 top
R36  10.86,13.97 180 top
R37  8.13,8.89 0 top
R38  8.13,9.91 0 top
R39  9.53,6.1 0 top
R40  3.68,12.32 180 top
R41  7.62,6.1 0 top
R42  3.68,11.31 180 top
R45  9.27,2.54 90 top
R46  26.42,6.86 90 top
R55  24.13,4.57 0 top
R56  26.42,9.4 90 top
R57  26.04,11.05 0 top
R58  22.23,8.77 90 top
R59  22.23,10.67 270 top
R60  34.54,10.67 90 top
R61  24.13,10.67 270 top
RST  21.59,1.4 180 top
SWD  46.99,1.27 90 top
TP1  6.35,17.78 180 bottom
TP2  6.35,19.69 180 bottom
TP3  6.35,21.59 180 bottom
TP4  12.57,4.7 0 bottom
U1  45.09,13.97 0 top
U2  21.59,15.12 270 top
U3  11.3,11.18 180 top
U4  15.88,20.96 0 top
U6  30.48,10.16 90 top
U7  30.48,6.86 90 top
U$8  [96BOARDS_IOT_EDITION_STANDARD]  0,0 0 top
U$48  [SEEED-SILK-280*268MIL]  39.05,19.43 0 bottom
U$49  [96BOARDS_SILK]  34.98,16.64 0 bottom
U$50  [OSHW_FILLX200_NOTEXT]  49.2,17.66 0 bottom
UART  36.83,1.27 90 top
USB  5,18.5 270 top
USR  27.94,1.4 180 top
USR1  1.78,13.34 180 top
X1  40.39,17.91 90 top
X2  51.82,19.05 90 top
X3  22.1,21.34 180 top

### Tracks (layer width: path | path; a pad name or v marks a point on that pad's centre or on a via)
!RESET
  Top 0.152: C13.2 D1.+ 49.47,9.88 R16.2 49.22,11.05 U1.24
BLE_!CTS  (via drill 0.25 pad 0.51)
  Top 0.152: U1.17 44.48,9.3 v45.28,8.51 | R13.2 R12.2 30.54,14.54 v30.48,14.48
  Route15 0.152: v45.28,8.51 44.13,7.37 38.73,7.37 31.62,14.48 v30.48,14.48 29.08,14.48 28.19,15.37 28.19,15.81 28.83,16.45 28.83,17.15 29.21,17.53 29.21,20.26 26.04,23.43 18.1,23.43 17.02,24.51 17.02,25.4 16.45,25.97 12.97,25.97 J1.3
BLE_!RTS  (via drill 0.25 pad 0.51)
  Top 0.152: U1.15 43.69,8.71 v43.88,8.51 | R9.2 30.54,17.78 | 30.54,17.78 R8.2 | v30.73,17.78 30.54,17.78
  Route15 0.152: v43.88,8.51 43.37,8 39.12,8 30.73,16.39 v30.73,17.78 30.73,19.62 26.29,24.07 21.53,24.07 21.02,24.58 21.02,25.47 20.45,26.04 19.04,26.04 J1.9
BLE_RX  (via drill 0.25 pad 0.51)
  Top 0.152: U1.18 44.88,9.6 v45.97,8.51 | J1.13 20.96,26.04 17.04,26.04 J1.7 | R15.2 28.51,17.78 | 28.51,17.78 R14.2 | v28.7,17.78 28.51,17.78
  Route15 0.152: v45.97,8.51 44.51,7.05 38.61,7.05 31.69,13.97 29.08,13.97 27.88,15.18 27.88,15.94 28.51,16.58 28.51,17.59 v28.7,17.78 28.7,20.32 25.91,23.12 17.89,23.12 J1.7
  Bottom 0.152: UART.2 36.83,3.37 37.59,4.13 41.59,4.13 v45.97,8.51
BLE_TX  (via drill 0.25 pad 0.51)
  Top 0.152: U1.16 44.09,9 v44.58,8.51 | J1.5 15.12,23.88 18.88,23.88 J1.11 | R10.2 28.51,15.62 | 28.51,15.62 R11.2 | v28.7,15.62 28.51,15.62
  Route15 0.152: v44.58,8.51 43.75,7.69 38.92,7.69 30.99,15.62 30.1,15.62 | J1.11 21.25,23.75 26.16,23.75 29.97,19.94 29.97,15.75 | 29.97,15.75 29.97,15.62 | v28.7,15.62 29.84,15.62 | 29.84,15.62 29.97,15.62 | 29.97,15.62 30.1,15.62 | 29.84,15.62 29.97,15.75 | 29.97,15.75 30.1,15.62
  Bottom 0.152: UART.1 37.47,4.45 41.47,4.45 44.58,7.56 v44.58,8.51
BUTTON/P0.27  (via drill 0.25 pad 0.51)
  Top 0.152: U1.39 46.48,17.4 46.86,17.78 47.12,17.78 47.5,18.16 v47.75,18.16 | R32.1 v35.56,5.08 33.66,3.18 29.97,3.18 29.61,2.82 USR.1
  Bottom 0.152: v47.75,18.16 47.5,18.16 35.56,6.23 v35.56,5.08
CH_STATU
  Top 0.152: U3.9 7.1,11.93 6.48,11.31 6.48,5.65 arc45 6.7,5.11 7.62,4.19 | R17.1 7.81,4 | 7.81,4 7.62,3.81 | 7.62,3.81 7.62,2.29 7.81,2.1 CHG.- | 7.62,4.19 7.81,4 | 7.62,3.81 7.62,4.19
DEBUG_!RST  (via drill 0.25 pad 0.51)
  Top 0.152: U2.8 v19.3,17.66 | R5.2 v49.53,8.77
  Route15 0.152: 49.53,3.81 20.19,3.81 19.3,4.7 19.3,9.78 16.89,12.19 16.89,15.24 v19.3,17.66 | 49.53,3.81 SWD.5 | 49.53,3.81 v49.53,8.77
DEBUG_SWCLK  (via drill 0.25 pad 0.51)
  Top 0.152: R1.2 v53.47,8.77 | v18.29,5.72 18.92,5.72 20.19,6.99 20.19,11.43 20.34,11.58 U2.18
  Route15 0.152: SWD.3 45.09,3.18 19.94,3.18 18.29,4.83 v18.29,5.72
  Bottom 0.152: v53.47,8.77 53.47,6.92 49.09,2.54 48.26,2.54 SWD.3
DEBUG_SWDIO  (via drill 0.25 pad 0.51)
  Top 0.152: R3.2 v53.47,10.8 | U2.17 19.84,7.4 v18.8,6.35
  Route15 0.152: SWD.4 47.31,3.5 20.07,3.5 18.8,4.77 v18.8,6.35
  Bottom 0.152: v53.47,10.8 53.98,10.29 53.98,6.99 49.53,2.54 SWD.4
GND  (via drill 0.25 pad 0.51, 0.64 pad 1.27)
  Top 0.152: v51.94,12.77 51.56,13.15 49.66,13.15 49.4,13.4 48.9,13.4 | Q3.2 8.38,6.42 R41.2 | v27.43,16.7 v29.46,16.7 29.53,16.64 29.65,16.64 | v27.43,16.7 27.5,16.64 27.62,16.64 | v27.43,16.7 v26.8,16.7
  Top 0.203: U3.13 10.55,10.37 v10.79,10.61
  Top 0.229: 46.35,13.96 46.57,14.17 U1.31 48.97,14.17 49.47,14.67 C7.1 50.05,14.66 | v45.02,18.42 44.58,17.97 C14.2 44.09,17.74 U1.45 44.09,14.97 U1.PAD
  Top 0.254: U3.8 10.55,12.18 10.79,11.94 v10.79,11.75 | 11.05,11.43 U3.PAD 11.3,11.24 v11.81,11.75 11.55,12.01 U3.6 | C21.2 19.88,20.13 20.45,19.56 v20.7,19.56 | R18.1 9.53,4 10.16,3.37
  Top 0.305: U3.10 9.14,11.43 | 9.14,11.43 8.63,11.43 C26.1 | U3.6 11.55,13.72 R36.1 | C31.1 13.4,22.16 C22.1 12.32,22.23 v11.43,23.12 | 9.14,11.43 8.64,10.92 7.49,10.92 v7.37,10.8
  Top 0.406: C29.- 13.72,14.48 13.34,14.86 v13.08,14.86 | R11.1 27.62,16.64 R15.1 | R13.1 29.65,16.64 R9.1
  Top 0.61: BAT.- 13.51,8.15 C30.1 | C38.1 28.43,9.4 v28.7,9.13
  other vias: 13.34,17.91 18.16,18.54 11.3,11.18 22.1,22.29 25.27,21.97 39.75,21.72 51.69,15.88 50.8,14.66 21.59,15.1 45.09,13.97 13.84,15.75 15.37,15.75 11.56,17.4 13.84,17.4 7.62,27.31 8.26,26.04 7.62,24.77 51.44,26.67 52.7,26.67 52.7,25.4 51.44,25.4 52.7,22.86 51.44,22.86 53.85,20.32 4.19,15.5 0.7,11.31 12.06,16.89 5.59,16.51 4.95,15.5 4.19,14.73 4.95,14.73 51.44,14.67 52.07,14.67 52.07,15.31 52.58,12.77 53.21,12.77 53.85,12.77 51.69,16.51 53.85,12.07 51.44,21.59 52.7,21.59 53.85,14.61 4.19,22.35 4.95,22.35 4.95,21.47 4.19,21.47 1.52,19.5 1.52,17.47 29.21,1.26 26.67,1.26 22.86,1.26 21.59,1.26 20.32,1.26 17.78,1.26 15.87,1.26 13.97,1.26 12.06,1.26 10.16,1.26 6.98,1.26 25.27,22.48 43.81,21.58 7.37,11.43 17.02,10.29 17.02,9.65 17.02,9.02 17.02,8.38 17.65,9.27 18.29,9.27 21.59,22.29 21.59,16.37 20.32,16.37 20.32,15.1 20.32,13.83 21.59,13.83 22.99,13.83 22.99,15.1 22.99,16.37 13.4,8.89 10.79,6.35 11.43,6.35 25.78,13.58 11.56,14.86 14.29,22.29 10.16,23.12 15.62,20.58 15.62,19.94 7.62,17.27 53.85,19.05 53.85,17.78 53.85,16.51 53.85,15.24 54.61,8.89 56.52,6.99 52.7,7.62 51.44,7.62 50.16,7.62 50.16,5.08 48.9,5.08 48.9,7.62 46.35,7.62 47.62,5.08 46.35,5.08 45.09,5.08 43.81,5.08 41.27,5.08 40.01,5.72 13.97,5.08 48.9,6.73 50.16,6.73 51.44,6.73 54.61,11.43 54.61,12.7 55.88,11.43 55.88,12.7 57.78,12.7 59.05,12.7 54.61,10.16 58.42,6.1 59.31,6.73 38.99,8.89 42.16,8.51 45.09,21.59 46.35,21.59 47.62,21.59 8,7.37 14.61,6.35 15.24,6.35 11.43,5.08 11.43,4.45 10.35,3.24 44.58,14.48 45.59,14.48 45.59,13.46 44.58,13.46 10.16,8.89 10.79,8.26 11.43,7.62 38.73,15.24 38.73,16.51 38.73,17.78 38.73,19.05 38.73,20.32 26.42,14.21 25.15,14.21 38.73,12.31 37.47,11.42 35.56,12.69 33.66,14.59 33.66,16.5 31.75,16.5 31.75,18.4 33.66,18.4 33.66,20.31 31.75,20.31 33.66,22.21 31.75,22.21 29.21,22.21 26.04,22.21 26.29,20.18 27.3,20.18 27.94,13.32 30.48,13.32 32.38,12.18 27.94,12.05 25.78,12.05 24.13,11.8 30.61,9.13 33.91,9.01 35.05,9.07 28.7,5.83 30.61,5.83 32.38,5.83 26.29,4.43 21.72,4.43 20.95,4.82 28.57,4.69 30.61,4.43 23.11,9.39 21.46,7.48 21.34,5.7 8.26,23.12 6.73,23.12 7.62,20.07 10.16,20.07 11.43,20.07 6.1,22.74
  pour Top (isolate 0.203, rank 6): -0.64,30.48 53.98,30.48 53.98,13.08 60.33,13.08 60.33,-0.63 -0.64,-0.63
  pour GND (isolate 0.203, rank 6): -0.64,30.48 53.98,30.48 53.98,13.08 60.33,13.08 60.33,-0.63 1.27,-0.63 1.27,-1.27 -0.64,-1.27
  pour Route15 (isolate 0.203, rank 6): -0.64,30.48 53.98,30.48 53.98,13.08 60.33,13.08 60.33,-0.63 1.91,-0.63 1.91,-1.9 -0.64,-1.9
  pour Bottom (isolate 0.203, rank 6): -0.64,30.48 53.98,30.48 53.98,13.08 60.33,13.08 60.33,-0.63 2.54,-0.63 2.54,-2.54 -0.64,-2.54
  pour Top (isolate 0.203, rank 6, no thermals): -0.64,23.12 5.71,23.12 5.71,13.97 -0.64,13.97
  pour Bottom (isolate 0.203, rank 6, no thermals): -0.64,23.12 5.71,23.12 5.71,13.97 -0.64,13.97
  pour Top (isolate 0.203, rank 6, no thermals): 10.16,-1.27 10.16,4.45 16.51,4.45 16.51,2.29 31.75,2.29 31.75,-1.27
N$1
  Top 0.203: R6.1 40.01,10.11 arc-45 39.82,9.66 C4.1 39.88,9.59 40.14,9.33 arc-45 40.32,8.88 40.32,7.37 arc90 41.97,5.72 51.4,5.72 arc45 55.26,7.32 55.78,7.84 arc-45 56.23,8.03 NFC.GND2 NFC.GND1
N$2
  Top 0.152: 23.37,22.1 X3.1 | X3.1 24.45,22.23 C23.1 | U2.4 21.84,20.7 X3.1
N$3
  Top 0.229: U1.46 43.69,18.6 43.94,18.86 C14.1 44.96,19.5 46.86,19.5 L3.2
N$4
  Top 0.152: U2.5 21.34,19.94 X3.3 20.83,20.96 20.51,21.28 C24.1
N$5
  Top 0.229: U1.47 43.28,18.9 44.2,19.81 L2.1
N$6
  Top 0.203: U2.14 18.15,14.37 16.13,16.39 13.46,16.39 11.11,18.74 9.78,18.74 R26.1
N$7
  Top 0.203: U2.13 18.22,14.87 16.32,16.77 13.65,16.77 11.3,19.12 9.72,19.12 9.46,19.37 R27.1
N$8  (via drill 0.25 pad 0.51)
  Top 0.203: R25.1 R26.2 8.49,18.5 7.2,18.5 | USB.3 5.88,18.5 | 5.88,18.5 6.1,18.5 | 6.1,18.5 6.26,18.5 | 6.26,18.5 6.31,18.5 | 6.31,18.5 6.73,18.5 | 6.73,18.5 7.2,18.5 | D2.1 6.73,18.5 | 6.26,18.5 6.6,18.16 6.22,18.16 | 7.2,18.5 6.86,18.16 | v6.1,17.91 6.1,18.16 | 6.1,18.16 6.1,18.29 | 6.1,18.29 6.1,18.5 | 5.88,18.5 6.1,18.29 | 6.31,18.5 6.1,18.29 | 6.1,18.16 6.22,18.16 | 6.22,18.16 6.35,18.29
  Bottom 0.203: TP1.T 6.22,17.78 v6.1,17.91
N$9
  Top 0.152: CHG.+ R45.2
N$10
  Top 0.152: Q7.3 23.3,8.19 | 23.3,8.19 23.24,8.26 | 23.24,8.26 22.29,9.21 R58.2 | Q6.1 23.24,7.88 23.24,8.13 | 23.24,8.13 23.3,8.19 | 23.24,8.13 23.24,8.26
N$11  (via drill 0.25 pad 0.51)
  Top 0.203: 6.6,19.15 8.29,19.15 R27.2 | D3.1 6.64,19.12 6.6,19.15 | USB.2 6,19.15 | 6,19.15 v6.1,19.05 | 6.6,19.15 6,19.15
  Bottom 0.203: v6.1,19.05 6.1,19.43 TP2.T
N$12
  Top 0.152: U1.2 41.76,15.77 41.53,16 41.53,18.67 40.77,19.43 | X1.2 40.77,19.43 | C1.2 40.83,19.5 40.77,19.43
N$13
  Top 0.152: U1.3 C2.2 | C2.2 40.83,15.94 | 40.83,15.94 X1.1 | 40.83,15.94 41.02,16.13
  Top 0.229: C2.2
N$14
  Top 0.152: U1.34 48.45,15.37 49.09,16 49.09,17.97 C3.1 52.32,18.67 52.7,18.29 X2.1
N$15
  Top 0.152: U1.35 48.41,15.77 48.77,16.13 48.77,18.61 C5.1 50.74,19.62 50.93,19.81 X2.3
N$16  (via drill 0.25 pad 0.51)
  Top 0.152: CDC.- v0.7,10.29 | v16.51,5.72 17.14,5.08 18.73,5.08 20.51,6.86 20.51,11.24 21.08,11.81 21.53,11.81 21.84,12.13 U2.21
  Bottom 0.152: v16.51,5.72 8.64,5.72 4.06,10.29 v0.7,10.29
N$17
  Top 0.203: R7.1 41.02,10.11 arc45 41.21,9.66 C6.2 41.15,9.59 40.89,9.33 arc45 40.7,8.88 40.7,7.37 arc90 41.97,6.1 51.36,6.1 arc45 54.95,7.59 56.08,8.71 arc45 56.26,9.16 NFC.D
N$18
  Top 0.203: U1.11 40.95,12.17 arc45 40.5,11.99 R6.2
N$19
  Top 0.229: C10.1 41.91,16.42 | 41.91,16.42 U1.1 | 41.91,16.42 41.91,16.29 42,16.2
N$20
  Top 0.152: U1.32 48.54,14.57 49.66,15.69 C11.1
N$21
  Top 0.152: C12.1 49.72,16.7 49.4,16.39 49.4,15.88 48.5,14.97 U1.33
N$22
  Top 0.203: U1.12 41.56,11.77 arc45 41.11,11.59 R7.2
N$25
  Top 0.203: L1.1 C7.2 U1.30
N$26
  Top 0.203: L1.2 C8.2 C9.2 58.57,13.78 ANT1.ANT
N$28
  pour Top (isolate 0.254, no thermals): 30.1,11.31 30.1,9.65 26.04,9.65 26.04,11.43 26.16,11.56 29.84,11.56
N$32
  Top 0.229: L3.1 45.91,20.51 L2.2
N$33
  Top 0.152: USR1.+ R35.2
N$34
  Top 0.152: BT.+ R40.2
N$35  (via drill 0.25 pad 0.51)
  Top 0.152: Q2.3 v9.78,7.62 | v0.7,13.34 USR1.-
  Bottom 0.152: v9.78,7.62 4.06,13.34 v0.7,13.34
N$36  (via drill 0.25 pad 0.51)
  Top 0.152: v0.7,12.32 BT.- | Q3.3 7.3,8.07 v6.99,8.38
  Bottom 0.152: v0.7,12.32 3.05,12.32 3.3,12.07 v6.99,8.38
N$39
  Top 0.203: Q1.3 9.78,17.08 R25.2
N$40  (via drill 0.25 pad 0.51)
  Top 0.203: 4.96,19.83 5.08,19.94
  Top 0.305: USB.1 5.07,19.8 5.21,19.94 5.08,19.94
  Top 0.61: F1.2 7.56,21.02 D4.2 6.29,21.02 v6.22,20.96 5.21,19.94
  Bottom 0.61: v6.22,20.96 6.22,21.47 TP3.T
N$41
  Top 0.152: U2.9 18.06,16.87 16.45,18.48 R23.2 R22.2
N$42
  Top 0.152: R28.2 CDC.+
N$43
  Top 0.152: R30.2 DAP.+
N$44
  Top 0.152: R29.2 MSD.+
N$46  (via drill 0.25 pad 0.51)
  Top 0.152: U2.7 20.34,18.14 20.07,18.42 19.05,18.42 v18.41,17.78 | v0.7,8.26 MSD.-
  Route15 0.152: v18.41,17.78 17.91,17.27 16,17.27 14.86,18.42 11.49,18.42 MSD.- v0.7,8.26
N$47  (via drill 0.25 pad 0.51)
  Top 0.152: DAP.- v0.7,9.27 | U2.12 18.55,15.37 18.29,15.62 18.29,16.19 16.7,17.78 v16.19,17.78
  Route15 0.152: v0.7,9.27 1.91,9.27 11.43,18.8 14.92,18.8 15.94,17.78 v16.19,17.78
N$58
  Top 0.152: R42.2 PWR.+
N$84
  pour Top (isolate 0.203, no thermals): 12.45,12 13.78,12 14.48,12.7 15.11,12.7 15.11,10.92 14.48,10.92 14.03,11.37 12.45,11.37
N$88
  Top 0.203: U3.7 11.05,13.21 10.41,13.85 R36.2 R34.1
N$89
  Top 0.152: U3.11 9.4,10.93 9.14,10.67 9.14,10.04 9.02,9.91 R38.2
N$90
  Top 0.152: U3.12 9.54,10.43 9.46,10.35 9.46,9.34 9.02,8.89 R37.2
N$91
  Top 0.305: U3.5 12.05,13.2 12.32,13.46 R33.1
P0.02  (via drill 0.25 pad 0.51)
  Top 0.152: U1.4 41.39,14.97 41.15,14.73 37.4,14.73 v35.5,16.64
  Route15 0.152: v35.5,16.64 35.5,21.51 J1.23
P0.03  (via drill 0.25 pad 0.51)
  Top 0.152: U1.5 41.49,14.57 41.34,14.42 36.77,14.42 v35.5,15.69
  Route15 0.152: J1.24 33.02,25.98 33.02,24.51 36.07,21.47 36.07,16.26 v35.5,15.69
P0.04  (via drill 0.25 pad 0.51)
  Top 0.152: U1.6 41.73,14.17 41.66,14.1 36.07,14.1 v35.5,14.67
  Route15 0.152: J1.25 34,24.39 36.45,21.94 36.45,15.62 v35.5,14.67
P0.05  (via drill 0.25 pad 0.51)
  Top 0.152: U1.7 35.99,13.77 v35.88,13.65
  Route15 0.152: J1.26 34.99,26.01 34.99,23.88 36.83,22.04 36.83,14.61 v35.88,13.65
P0.06  (via drill 0.25 pad 0.51)
  Top 0.152: U1.8 41.75,13.37 41.66,13.46 37.21,13.46 v36.39,12.64
  Route15 0.152: J1.27 36,23.37 37.21,22.16 37.21,13.46 v36.39,12.64
P0.07  (via drill 0.25 pad 0.51)
  Top 0.152: U1.9 41.64,12.97 41.48,13.13 37.58,13.13 v37.08,12.64
  Route15 0.152: J1.28 37.02,25.98 37.02,22.8 37.59,22.23 37.59,13.15 v37.08,12.64
P0.08  (via drill 0.25 pad 0.51)
  Top 0.152: U1.10 41.53,12.57 41.3,12.8 37.95,12.8 v37.78,12.64
  Route15 0.152: J1.29 38,12.86 v37.78,12.64
P0.11  (via drill 0.25 pad 0.51)
  Top 0.152: U1.14 43.28,8.62 v43.18,8.51
  Route15 0.152: J1.30 38.99,26.01 38.99,21.72 39.94,20.77 39.94,10.42 41.34,9.02 42.67,9.02 v43.18,8.51
P0.16  (via drill 0.25 pad 0.51)
  Top 0.152: U1.19 45.28,9.9 v46.67,8.51
  Route15 0.152: v46.67,8.51 45.85,9.34 41.47,9.34 40.26,10.54 40.26,24.74 J1.31
P0.17  (via drill 0.25 pad 0.51)
  Top 0.152: U1.20 45.69,10.2 v47.37,8.51
  Route15 0.152: J1.32 40.96,26.05 40.96,24.45 40.58,24.07 40.58,10.67 41.59,9.65 46.23,9.65 v47.37,8.51
P0.18  (via drill 0.25 pad 0.51)
  Top 0.152: U1.21 46.09,10.5 v47.37,9.21
  Route15 0.152: J1.33 40.89,23.9 40.89,10.8 41.72,9.97 46.61,9.97 v47.37,9.21
P0.19  (via drill 0.25 pad 0.51)
  Top 0.152: U1.22 46.48,10.6 47.12,9.97 47.31,9.97 v47.37,9.91
  Route15 0.152: J1.34 42.99,26.01 42.99,22.48 41.21,20.7 41.21,10.93 41.85,10.29 46.99,10.29 v47.37,9.91
P0.20/BLE_SDA  (via drill 0.25 pad 0.51)
  Top 0.152: U1.23 46.88,10.71 47.18,10.42 47.75,10.42 v47.88,10.54
  Route15 0.152: v47.88,10.54 47.82,10.61 41.97,10.61 41.53,11.05 41.53,20.58 45.02,24.07 45.02,27.56 44.32,28.26 27.81,28.26 26.99,27.43 26.99,25.97 26.97,25.97 J1.17
P0.22/BLE_SCL  (via drill 0.25 pad 0.51)
  Top 0.152: U1.27 48.39,12.57 48.96,12 50.86,12 v51.05,12.19
  Route15 0.152: v50.8,24.01 50.8,22.74 50.23,22.16 50.23,13.53 51.05,12.7 v51.05,12.19
  Bottom 0.152: v50.8,24.01 25,24.01 J1.15
P0.23/BLE_SPI_MOSI  (via drill 0.25 pad 0.51)
  Top 0.152: U1.28 48.43,12.97 49.09,12.32 50.16,12.32 v50.42,12.58
  Route15 0.152: v50.29,23.5 50.29,22.74 49.91,22.35 49.91,13.21 50.42,12.7 v50.42,12.58
  Bottom 0.152: J1.14 22.99,26.02 22.99,24.51 23.81,23.69 50.1,23.69 v50.29,23.5
P0.24/BLE_SPI_!SS  (via drill 0.25 pad 0.51)
  Top 0.152: U1.29 48.48,13.37 49.02,12.83 v49.28,12.83
  Route15 0.152: v49.78,22.99 49.78,22.74 49.59,22.55 49.59,13.15 v49.28,12.83
  Bottom 0.152: J1.12 21.02,25.98 21.02,24.51 22.16,23.37 49.4,23.37 v49.78,22.99
P0.25/BLE_SPI_MISO  (via drill 0.25 pad 0.51)
  Top 0.152: U1.37 47.56,16.9 v47.75,16.7
  Route15 0.152: v47.75,16.7 48.96,17.91 48.96,23.5 50.04,24.58 50.04,28.07 49.21,28.89 19.89,28.89 J1.10
P0.26/BLE_SPI_SCK  (via drill 0.25 pad 0.51)
  Top 0.152: U1.38 46.88,17.3 47.05,17.46 v47.75,17.46
  Route15 0.152: v47.75,17.46 48.07,17.46 48.64,18.04 48.64,23.62 49.72,24.7 49.72,27.94 49.09,28.58 20.07,28.58 18.99,27.5 18.99,26.55 18.48,26.04 16.96,26.04 J1.8
P0.28/BT_LED  (via drill 0.25 pad 0.51)
  Top 0.152: U1.40 46.09,17.45 46.74,18.1 46.99,18.1 v47.75,18.86 | Q3.1 7.37,6.29 R41.1 v7.18,5.46
  Bottom 0.152: v7.18,5.46 9.97,2.67 31.56,2.67 v47.75,18.86
P0.29/USR_LED  (via drill 0.25 pad 0.51)
  Top 0.152: U1.41 45.69,17.49 v47.05,18.86 | Q2.1 9.27,6.29 R39.1 9.08,5.72 9.27,5.53 10.28,5.53 10.67,5.14 10.67,4.7 v10.16,4.19
  Bottom 0.152: v10.16,4.19 11.37,2.99 31.43,2.99 47.05,18.61 v47.05,18.86
P0.30/AIN6  (via drill 0.25 pad 0.51)
  Top 0.152: R17.2 R18.2 v10.16,4.89 | U1.42 45.28,17.54 46.35,18.61 v46.35,18.86
  Bottom 0.152: v10.16,4.89 11.75,3.3 31.3,3.3 46.35,18.35 v46.35,18.86
P0.31/READ_VBAT  (via drill 0.25 pad 0.51)
  Top 0.152: R19.2 v34.54,7.5 C18.1 R20.1 | U1.43 44.88,17.58 45.66,18.35 v45.66,18.86
  Bottom 0.152: v34.54,7.5 35.05,7.5 45.66,18.1 v45.66,18.86
PROG-!CTS!  (via drill 0.25 pad 0.51)
  Top 0.152: v19.24,11.88 19.05,12.07 U2.16 | R8.1 29.08,18.86 27.24,18.86 25.91,17.53 v25.27,17.53
  Route15 0.152: v25.27,17.53 24.13,16.39 24.13,13.34 21.59,10.8 20.32,10.8 v19.24,11.88
PROG-!RTS!
  Top 0.152: U2.30 25.92,15.87 27.24,14.54 29.08,14.54 R12.1
PROG-BUTTON  (via drill 0.25 pad 0.51)
  Top 0.152: U2.3 22.34,18.28 v22.35,18.29 | RST.2 19.91,5.82 20.83,6.73 20.83,10.8 v21.34,11.31
  Route15 0.152: v21.34,11.31 23.75,13.72 23.75,16.89 v22.35,18.29
PROG-RESET
  Top 0.152: C19.2 R21.1 23.62,19.18 22.84,18.4 U2.2
PROG-RX
  Top 0.152: U2.31 25.93,16.37 27.18,15.12 R10.1
PROG-TX
  Top 0.152: U2.32 26.01,16.87 27.43,18.29 R14.1
PROG_VCC  (via drill 0.25 pad 0.51)
  Top 0.203: R29.1 R30.1 R28.1 4.83,10.29 6.73,12.19 6.73,15.24 | v6.22,15.31 R24.2 6.73,15.24 | R21.2 25.46,18.86 24.77,18.16 v24.38,18.16 | Q1.2 6.86,15.12 6.73,15.24
  Top 0.254: U2.6 20.84,18.53 20.13,19.24 C21.1
  Top 0.279: U2.29 24.96,15.37 v25.15,15.18 25.18,15.15
  Top 0.406: C32.2 18.29,19.43 v18.8,18.93 19.37,18.93 C21.1 | C20.1 25.21,15.12 25.18,15.15
  Top 0.61: U4.2 18.2,19.9 C32.2
  Route15 0.203: v18.8,18.93 18.54,19.18 8.38,19.18 6.99,17.78 6.99,16.07 v6.22,15.31
  Bottom 0.406: v18.8,18.93 23.62,18.93 v24.38,18.16 24.38,15.94 v25.15,15.18
PWR_!BTN  (via drill 0.25 pad 0.51)
  Top 0.152: Q7.1 24.64,9.72 R61.2 23.18,11.18 v22.86,11.18 22.8,11.12 R59.1
  Route15 0.152: J1.4 11.05,26.05 11.05,24.45 12.7,22.8 23.69,22.8 25.78,20.7 25.78,17.02 24.51,15.75 24.51,13.21 22.86,11.56 v22.86,11.18
RST_!BTN  (via drill 0.25 pad 0.51)
  Top 0.152: v50.42,9.78 D1.- 50.97,8.79 R5.1
  Route15 0.152: v50.42,9.78 50.93,9.78 51.31,10.16 51.31,11.05 50.93,11.43 49.78,11.43 48.77,12.45 48.77,17.27 49.28,17.78 49.28,23.37 50.35,24.45 50.35,28.2 49.34,29.21 16.21,29.21 J1.6
SWDCLK
  Top 0.152: R1.1 R2.2 51.44,10.35 51.44,11.18 51.24,11.37 48.7,11.37 48.3,11.77 U1.25
SWDIO
  Top 0.152: R3.1 R4.2 51.56,11.81 51.44,11.69 48.83,11.69 48.35,12.17 U1.26
USB5V  (via drill 0.25 pad 0.51)
  Top 0.152: 15.88,6.86 15.88,5.84 11.81,1.78 10.41,1.78 10.1,2.1 R45.1 | 15.88,6.86 15.49,7.24 | 15.88,6.86 16.26,7.24
  Top 0.203: R34.2 8.38,13.91 C26.2
  Top 0.305: U3.2 13.59,10.93 13.84,10.67
  Top 0.61: 13.72,20.45 C31.2 12.57,20.45 12.32,20.7 C22.2 11.24,21.28 F1.1 | 13.72,20.45 14.99,21.72 15.75,21.72 15.88,21.85 U4.3 | 13.72,20.45 13.72,19.24 R22.1 14.41,17.97 v14.61,17.78 | 13.84,10.67 14.48,10.04 C25.2 C27.2 v14.61,7.62 14.99,7.24 15.49,7.24 16.26,7.24 16.95,7.24 R31.1 | v9.4,12.83 8.38,12.83 C26.2
  Route15 0.203: 14.1,12.83 14.61,12.83
  Route15 0.406: v44.32,22.48 46,24.16 J1.37
  Route15 0.61: 14.1,12.83 14.48,13.21 | 14.1,12.83 14.48,12.45 | v14.61,7.62 14.61,12.83 v14.61,17.78 | v9.4,12.83 14.1,12.83
  Bottom 0.406: v14.61,17.78 17.84,21.02 40.96,21.02 42.42,22.48 v44.32,22.48
USB_!CONNECT!
  Top 0.152: U2.15 17.76,13.87 16.76,14.86 13.97,14.86 13.4,15.43 10.6,15.43 10.16,14.99 9.27,14.99 8.89,15.37 8.89,16.13 8.64,16.39 Q1.1 6.92,16.39 R24.1
VBAT  (via drill 0.25 pad 0.51)
  Top 0.152: R19.1 32.51,3.88 29.08,3.88 27.94,2.73 v27.94,1.91
  Top 0.279: U3.14 11.05,9.15 11.31,8.89 11.8,8.89 | U3.16 12.05,9.15 11.8,8.89 | v12.51,8.89 12.57,8.89 | 11.8,8.89 v12.51,8.89 | 12.05,9.35 v12.51,8.89
  Top 0.61: v12.51,8.89 C30.2 12.49,8.24 BAT.+ 12.49,5.67 v13.21,4.96
  Route15 0.203: v12.51,8.89 12.51,4.45 15.05,1.91 v27.94,1.91
  Bottom 0.61: TP4.T 12.95,4.7 v13.21,4.96
VCC  (via drill 0.25 pad 0.51)
  Top 0.152: R16.1 v50.8,10.8
  Top 0.203: U1.48 42.88,18.52 v42.61,18.8 42.93,19.12 C17.1
  Top 0.229: U1.13 42.88,11.01 | U1.13 42.88,10.31 C15.1 | U1.36 48.24,16.17 48.39,16.32 48.39,18.8 48.77,19.18 C16.1 v48.13,19.62 | U1.13 42.23,11.05 v42.16,11.12
  Top 0.406: v33.15,8.26 C41.2 32.96,7.81 U7.2 | R32.2 36.51,6.8 v36.83,6.48 36.83,6.35 SWD.1 | R60.1 33.97,10.23 v33.91,10.16
  Route15 0.152: v50.8,10.8 50.55,11.05 42.23,11.05 v42.16,11.12
  Route15 0.406: v42.61,18.8 42.61,16.39 42.16,15.94 v42.16,11.12 | v33.15,8.26 33.15,8 34.67,6.48 v36.83,6.48
  Bottom 0.406: v42.61,18.8 42.55,18.8 43.37,19.62 v48.13,19.62 | v42.16,11.12 37.53,6.48 v36.83,6.48 | v33.15,8.26 33.15,9.4 v33.91,10.16
VCC2
  Top 0.61: 34.16,11.18 34.23,11.12 R60.2 34.54,11.56
  Top 0.813: U6.2 32.96,11.11 C39.2 33.4,11.18 34.16,11.18 | 34.54,11.56 34.54,20.07 37.47,22.99 41.99,22.99 J1.35
VIN  (via drill 0.25 pad 0.51)
  Top 0.279: U3.15 11.55,10.09 11.89,10.43 U3.1 13.07,10.43 13.46,10.04 v13.46,9.78
  Top 0.61: R31.2 19.14,8.54 19.14,10.83 18.41,11.56 18.16,11.56 C28.2 | R59.2 21.65,10.23 v21.46,10.04 21.4,9.97 21.4,8.57 21.65,8.32 R58.1 22.23,6.23 22.73,5.72 Q6.2 23.69,5.27 R55.1
  Route15 0.61: 18.03,11.94 17.53,12.45 v17.53,12.7 v18.03,12.7 18.03,11.94 | 18.03,11.94 19.94,10.04 20.83,10.04 | 20.83,10.04 v21.46,10.04 21.4,9.97 v21.4,9.46 20.83,10.04
  Bottom 0.61: v18.03,12.7 v17.53,12.7 17.27,12.7 v15.75,11.18 | v13.46,9.78 14.35,9.78 v15.75,11.18 | v15.75,11.18 15.81,11.24 | v21.4,9.46 21.4,9.97 v21.46,10.04
  pour Top (isolate 0.203, rank 2, no thermals): 15.49,14.35 16.76,14.35 18.67,12.45 18.67,10.92 15.49,10.92
VLOAD  (via drill 0.25 pad 0.51)
  Top 0.203: R42.1 R40.1 R35.1
  Top 0.254: v5.08,11.31 R42.1
  Top 0.406: U7.3 29.34,6.86 28.57,7.62 C40.2 v27.18,7.62 26.92,7.62 R46.2 R56.1
  Bottom 0.254: v5.08,11.31 9.4,6.99 16.13,6.99 19.43,3.69 23.24,3.69 v27.18,7.62
  pour Top (isolate 0.254, no thermals): 29.97,6.35 26.42,6.35 25.91,6.86 25.91,9.15 27.3,9.15 28.96,7.75 29.97,7.75 30.23,7.5 30.23,6.61
VSUPPLY
  Top 0.406: 25.53,10.99 R57.1
  Top 0.61: R55.2 24.57,5.91 Q6.3
  Top 0.813: R46.1 25.27,6.1 Q6.3 25.4,6.73 | 25.53,10.99 25.53,10.92 25.4,10.8 25.4,6.73 | 25.4,6.73 25.91,6.23

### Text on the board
tNames: 2 | 40 | 1 | 39 | + | - | TX | RX | GND | 1V8 | GND | CLK | DIO | !RST
bNames: BLE Nitrogen | v1.1 by Seeed & 96Boards | 02/16/2017
dxf: F | F | F | F | F | F | F | F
